(* Logix 5000 AddOnInstructionDefinition export Banner_Q5X_Jam_Param_v4; software revision 33.00 *)

TYPE Banner_BDC_v4 :   // UDT that covers all of the data for BDC options.
STRUCT
   SP1 : DINT;
   SP2 : DINT;   // In FGS, defines the second switching point. Other modes do not use this parameter.
   Switchpoint_Logic : SINT;   // 0 = Light Operate, 1 = Dark Operate
   BDC_Mode : INT;   // 132 = Jam Retroreflective, 133 = Jam Background Suppression
   Hysteresis : INT;   // Hysteresis value for the switchpoint. A value of 0 will result in automatically calculated hysteresis
   Delay_Mode : SINT;   // 0 = Disabled, 1= On-Off Delay, 2 = Oneshot, 3 = Totalizer
   Delay_Time_1 : DINT;   // 0 to 90000
   Delay_Time_2 : DINT;   // 0 to 90000
   BGS_Teach_Offset_Mode : SINT;   // 0 = Auto, 1 = User Selected
   FGS_Window_Size_Mode : SINT;   // 0 = Auto, 1 = User Selected
   User_Teach_Offset : INT;   // User selected teach offset. In FGS or BGS mode this value can be either positive or negative. In BGS mode, this mode must be set to 0 if the Teach Offset Mode is set to Auto. In all other teach modes this value must be written as 0.
   FGS_User_Window_Size : INT;   // In FGS mode this will set the size of the window for a teach. If teach offest mode is set to Auto, this value must be written as 0. In all other teach modes this value must be set to 0.
   Teach_Minimum_Moving_Range : DINT;   // Teach minimum moving range.
   Teach_Jam_Detection_Response_Time : DINT;   // Teach Jam detection response time.
   BDC_AutoThresholding : SINT;   // 0 = On, 1 = Off, 2 = High Speed. Set the auto-thresholding mode (dual teach mode only).
END_STRUCT
END_TYPE

TYPE Banner_IOL_Port_v4 :   // UDT that has all of the data items necessary to communicate with a specific Port on a IO-Link Master
STRUCT
   Port_Controlled : INT;   // Each bit represents a port on an IO-Link Master. Set to 1 to tell AOI to control that port.
   Port_Activate : INT;   // Each bit represents a port on an IO-Link Master. When ON that port will process any commands in queue.
   Port_Read : INT;   // Each bit represents a port on an IO-Link Master. Used to determine when device AOI has requested a Read command.
   Port_Write : INT;   // Each bit represents a port on an IO-Link Master. Used to determine when device AOI has requested a Write command.
   Port_RW_Complete : INT;   // Each bit represents a port on an IO-Link Master. Tells device AOI that Read or Write request has been completed.
   Port_Device_Read : INT;
   Data_Transfer : SINT[190];   // Array to transfer data from IO-Master to device AOIs.
END_STRUCT
END_TYPE

TYPE Banner_Q5X_Jam_RD_v4 :   // UDT that stores the Write Data for a Q5X.
STRUCT
   Master_Cycle_Time : INT;
   Min_Cycle_Time : INT;
   M_Sequence_Capability : INT;
   IO_Link_Version_ID : INT;
   Process_Data_Input_Length : INT;
   Process_Data_Output_Length : INT;
   Combined_Vendor_ID : DINT;   // IO-Link Vendor ID
   Vendor_ID1 : INT;
   Vendor_ID2 : INT;
   Combined_Device_ID : DINT;   // IO-Link Device ID
   Device_ID1 : INT;
   Device_ID2 : INT;
   Device_ID3 : INT;
   Serial_Number : STRING;
   Teach_State : SINT;
   SP1_TP1 : SINT;
   SP1_TP2 : SINT;
   Measurement_1 : DINT;
   Excess_Gain : DINT;   // Amount of single measured over the minimum threshold.
   Stability : SINT;   // 0 = No target exists, 1 = Marginal or multiple peaks, 2 = Stable
   Multiple_Peak_State : SINT;   // 0 = Multiple peaks not present, 1 = Multiple peaks present
   Emitter_Status : SINT;   // 0 = Active, 1 = Inactive
   Laser_Fault_Status : SINT;   // 0 = No Fault, 1 = Fault Present
   BDC1_Totalizer_Counts : DINT;
   BDC2_Totalizer_Counts : DINT;
   All_Time_Run_Time : DINT;   // Read only counter that tracks the total time sensor has been running since manufacture. Value in Hours.
   Display : STRING;   // Last Display information
END_STRUCT
END_TYPE

TYPE Banner_Q5X_Jam_v4 :   // All of the parameters for a Q5X.
STRUCT
   Initial_Global_Read : BOOL;   // Determines if all of the IO-Link data has been read into the PLC yet
   Command : INT;   // Value placed in here will activate a read or write to a specifc IO-Link Index
   Read : Banner_Q5X_Jam_RD_v4;   // Read Only Data
   Write : Banner_Q5X_Jam_WD_v4;   // Write Data
   Archive : Banner_Q5X_Jam_WD_v4;   // Archive Data
   Reset : BOOL;   // Resets AOI. This will force a complete parameter read of the sensor.
END_STRUCT
END_TYPE

TYPE Banner_Q5X_Jam_WD_v4 :   // UDT that stores the Write Data for a Q5X.
STRUCT
   System_Command : INT;   // See IODD file for list of commands that can be activated via the System Command interface
   Parameter_Access_Lock : SINT;   // Write access to all parameters is prohibited while value is 1. Only this parameter can be adjusted when value is 1.
   Data_Storage_Lock : SINT;   // Automatic data storage is disabled when this value is equal to 1. Read access is not affected.
   Local_Parameterization_Lock : SINT;   // Parameterization via local control elements on device is disabled.
   Local_User_Interface_Lock : SINT;   // Operation of local user interface is disabled.
   Teach_in_Channel : SINT;   // 0 = Default, 1 = BDC1, 2 = BDC2
   BDC : Banner_BDC_v4[3];
   Response_Speed : SINT;   // 2 = 15ms, 3 = 25ms, 4 = 50ms
   Gain : SINT;   // 0 = High excess gain mode, 1 = Standard excess gain mode
   Secondary_Output_Mode : SINT;   // 0 = Remote Teach Input, 1 = Laser On, 2 = Master, 3 = Slave, 4 = Complementary Output, 5 = Laser Off, 6 = Pulse Freq Modulation, 7 = Independent Output
   Zero_Reference_Location : SINT;   // 0 = Near, 1 = Far
   Shift_Zero_after_Teach : SINT;   // 0 = Off, 1 = On
   Display_Read : SINT;   // 0 = On, 1 = On Inverted, 2 = Off, 3 = Off Inverted
   Pushbutton_Lockout : SINT;   // 0 = No Lockout, 1 = Pushbuttons Locked, 2 = Operator Lockout
   Output_Polarity : SINT;   // 0 = Default, 1 = PNP, 2 = NPN
   IOL_Filter_Time : INT;   // Time to average IOl process data measurement between updates
   Include_Binary : SINT;   // 0 = Include, 1 = Don't Include
   Measurement_1 : SINT;   // 0 = Disabled, 1 = Excess Gain, 2 = Excess Gain / 10
   Measurement_2 : SINT;   // 0 = Disabled, 1 = Distance Value, 2 = Displayed Distance, 3 = Channel 2 Dual Mode Percent
   Resettable_Run_Time : DINT;
   PFM_Near : DINT;   // 100 to 45000 in Hz
   PFM_Far : DINT;   // 100 to 45000 in Hz
   All_Time_Run_Time_Event_Time : DINT;
   Resettable_Run_Time_Event_Time : DINT;
END_STRUCT
END_TYPE

ADD_ON_INSTRUCTION Banner_Q5X_Jam_Param_v4   (* revision 4.0, vendor Banner Engineering *)
// AOI to read and write parameter data to an IO-Link Q5X.
VAR_IN_OUT
   Q5X : Banner_Q5X_Jam_v4; {required}
   Port_Data : Banner_IOL_Port_v4; {required}
END_VAR
VAR_INPUT
   Port : DINT; {required}
END_VAR
VAR
   Local_Control : DINT; {access None}
   Global_Read_Command_Value : INT; {access None}
   Global_Write_Command_Value : INT; {access None}
   Command_Being_Processed : BOOL; {access None}
   Update_Archive : BOOL; {access None}
   Index_Write_Inprocess : INT; {access None}
   Index_Write_Control : INT; {access None}
   Inprocess_Index : DINT; {access None}
END_VAR

ROUTINE Logic   (* ladder *)
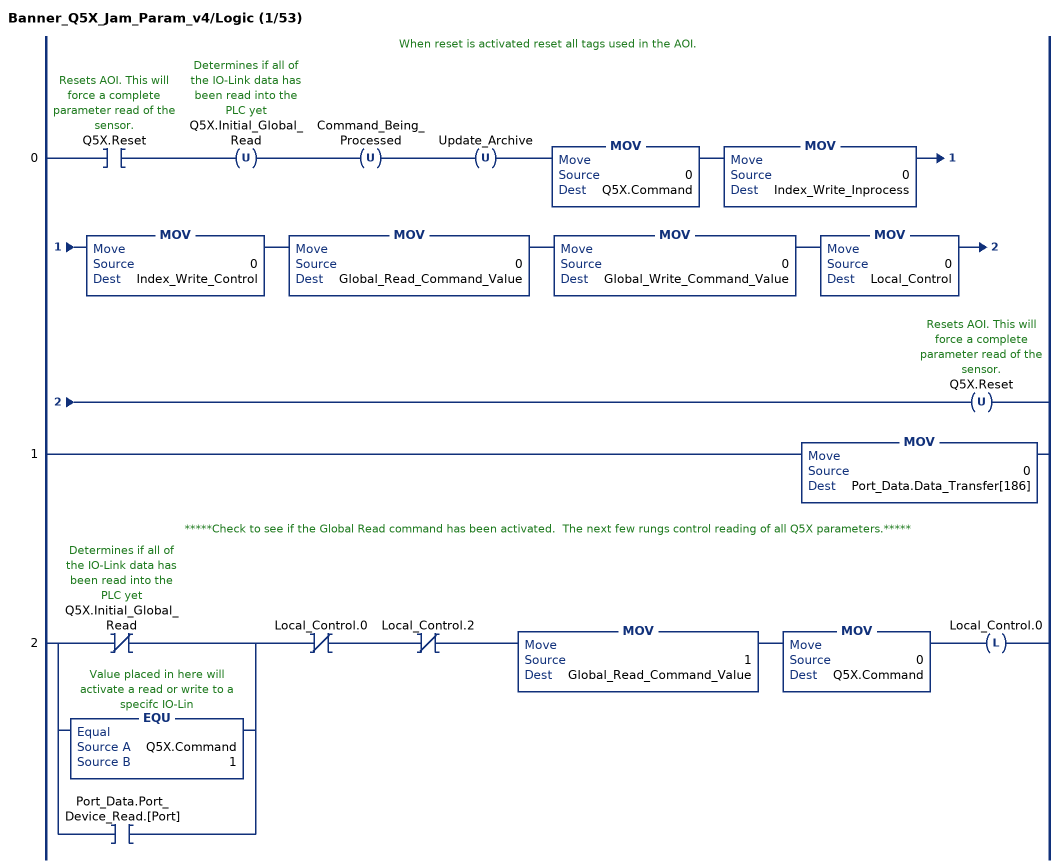
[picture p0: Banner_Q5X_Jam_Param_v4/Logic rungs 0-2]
   // When reset is activated reset all tags used in the AOI.
   0: XIC(Q5X.Reset)OTU(Q5X.Initial_Global_Read)OTU(Command_Being_Processed)OTU(Update_Archive)MOV(0,Q5X.Command)MOV(0,Index_Write_Inprocess)MOV(0,Index_Write_Control)MOV(0,Global_Read_Command_Value)MOV(0,Global_Write_Command_Value)MOV(0,Local_Control)OTU(Q5X.Reset);
   1: MOV(0,Port_Data.Data_Transfer[186]);
   // *****Check to see if the Global Read command has been activated.  The next few rungs control reading of all Q5X parameters.*****
   2: [XIO(Q5X.Initial_Global_Read) ,EQU(Q5X.Command,1) ,XIC(Port_Data.Port_Device_Read.[Port]) ]XIO(Local_Control.0)XIO(Local_Control.2)MOV(1,Global_Read_Command_Value)MOV(0,Q5X.Command)OTL(Local_Control.0);
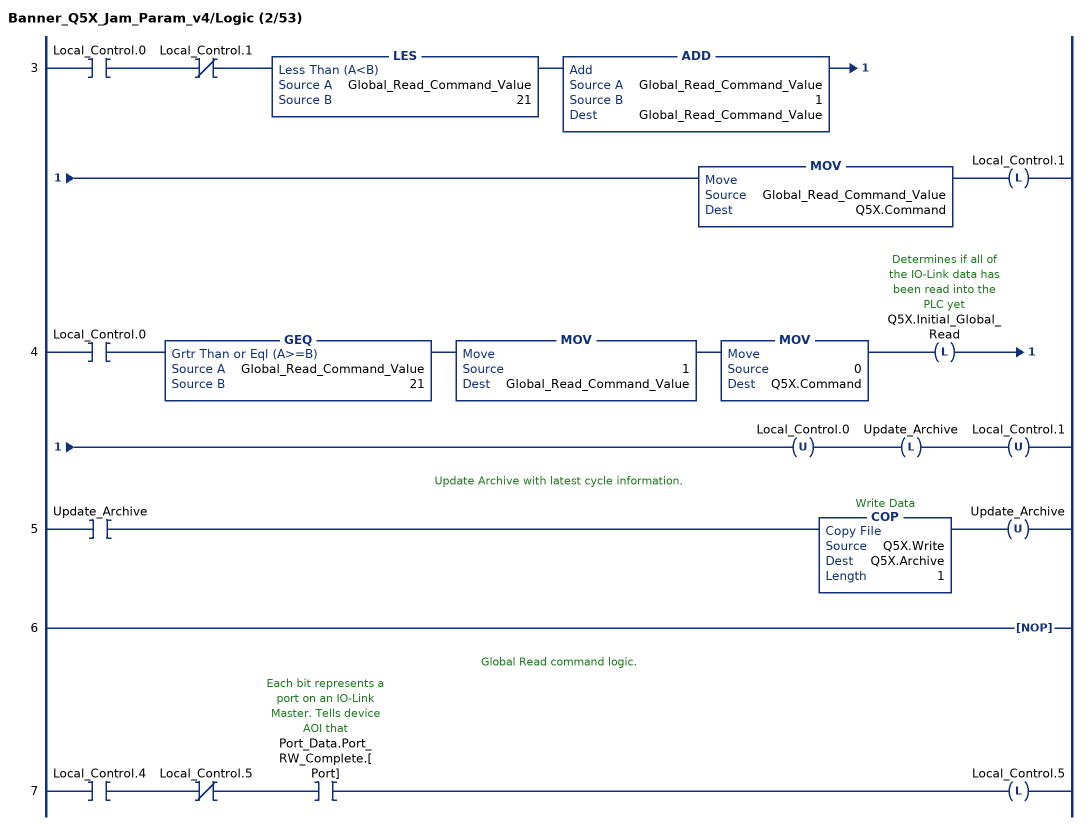
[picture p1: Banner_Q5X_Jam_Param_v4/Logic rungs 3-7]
   3: XIC(Local_Control.0)XIO(Local_Control.1)LES(Global_Read_Command_Value,21)ADD(Global_Read_Command_Value,1,Global_Read_Command_Value)MOV(Global_Read_Command_Value,Q5X.Command)OTL(Local_Control.1);
   4: XIC(Local_Control.0)GEQ(Global_Read_Command_Value,21)MOV(1,Global_Read_Command_Value)MOV(0,Q5X.Command)OTL(Q5X.Initial_Global_Read)OTU(Local_Control.0)OTL(Update_Archive)OTU(Local_Control.1);
   // Update Archive with latest cycle information.
   5: XIC(Update_Archive)COP(Q5X.Write,Q5X.Archive,1)OTU(Update_Archive);
   6: NOP();
   // Global Read command logic.
   7: XIC(Local_Control.4)XIO(Local_Control.5)XIC(Port_Data.Port_RW_Complete.[Port])OTL(Local_Control.5);
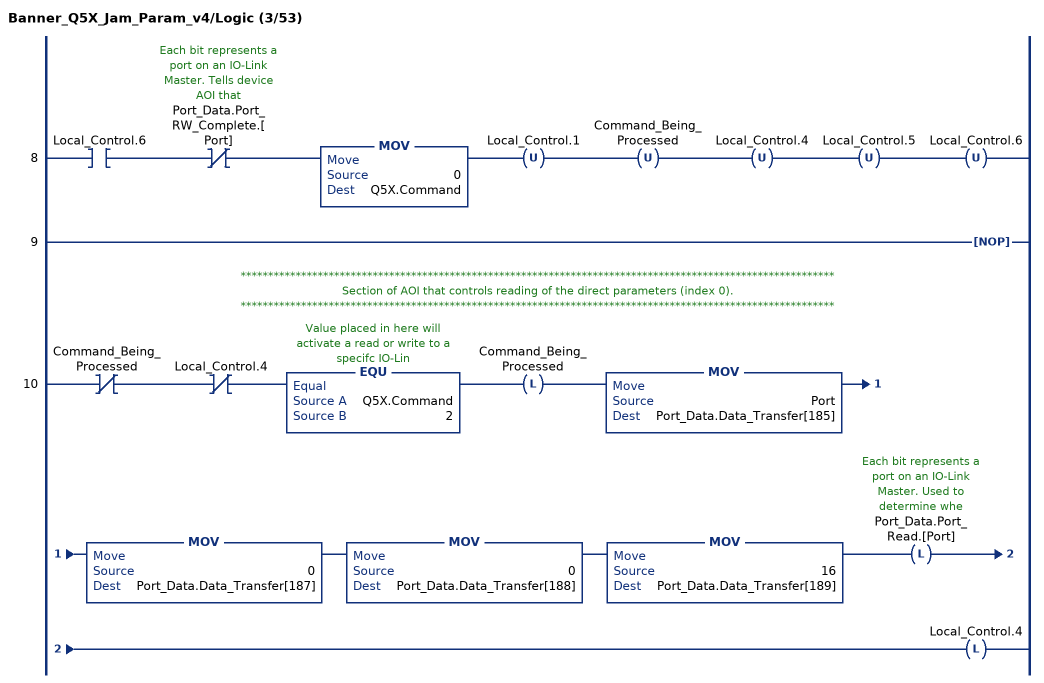
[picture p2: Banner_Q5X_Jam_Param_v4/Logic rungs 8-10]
   8: XIC(Local_Control.6)XIO(Port_Data.Port_RW_Complete.[Port])MOV(0,Q5X.Command)OTU(Local_Control.1)OTU(Command_Being_Processed)OTU(Local_Control.4)OTU(Local_Control.5)OTU(Local_Control.6);
   9: NOP();
   // ************************************************************************************************************
   // Section of AOI that controls reading of the direct parameters (index 0).
   // ************************************************************************************************************
   10: XIO(Command_Being_Processed)XIO(Local_Control.4)EQU(Q5X.Command,2)OTL(Command_Being_Processed)MOV(Port,Port_Data.Data_Transfer[185])MOV(0,Port_Data.Data_Transfer[187])MOV(0,Port_Data.Data_Transfer[188])MOV(16,Port_Data.Data_Transfer[189])OTL(Port_Data.Port_Read.[Port])OTL(Local_Control.4);
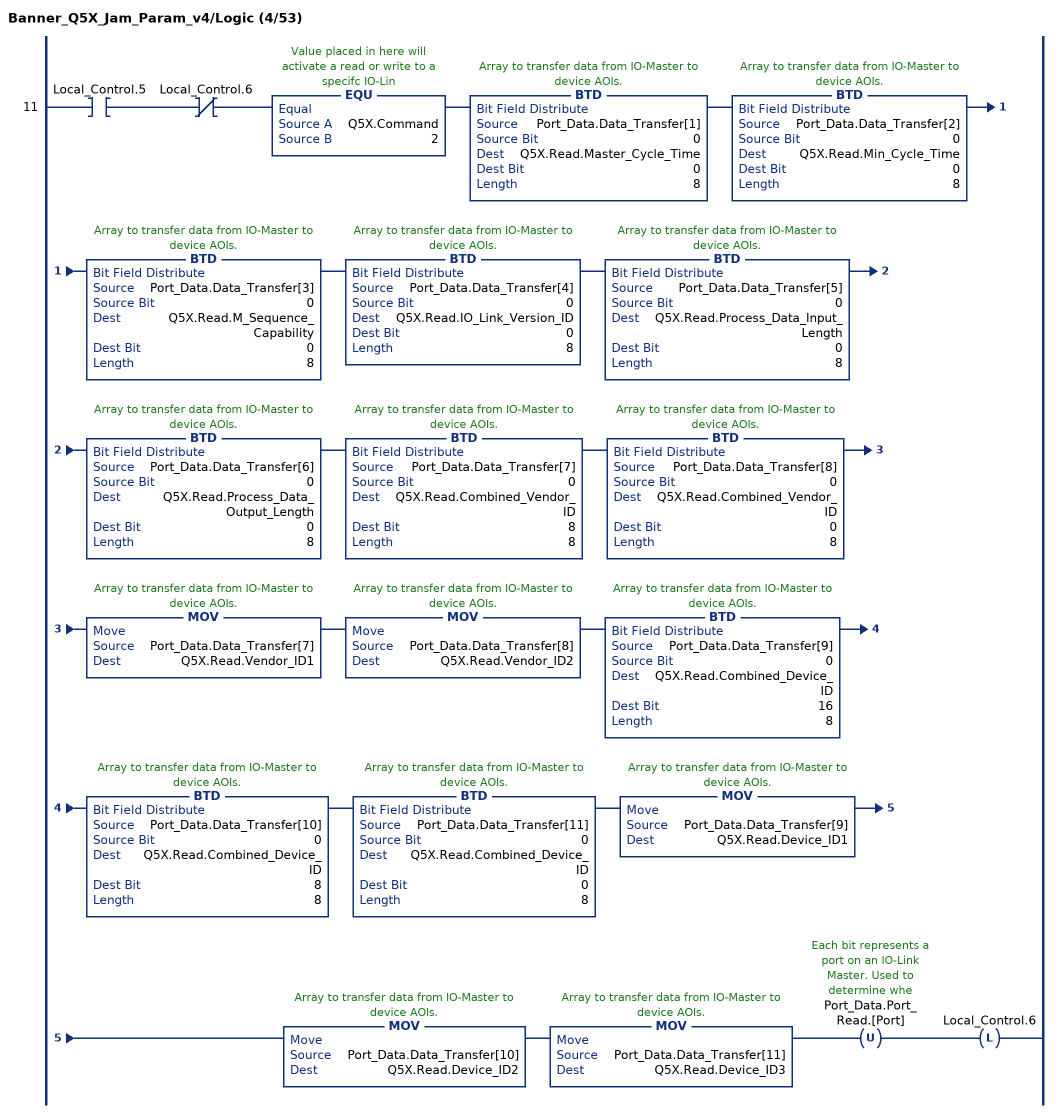
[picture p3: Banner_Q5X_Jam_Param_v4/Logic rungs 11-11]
   11: XIC(Local_Control.5)XIO(Local_Control.6)EQU(Q5X.Command,2)BTD(Port_Data.Data_Transfer[1],0,Q5X.Read.Master_Cycle_Time,0,8)BTD(Port_Data.Data_Transfer[2],0,Q5X.Read.Min_Cycle_Time,0,8)BTD(Port_Data.Data_Transfer[3],0,Q5X.Read.M_Sequence_Capability,0,8)BTD(Port_Data.Data_Transfer[4],0,Q5X.Read.IO_Link_Version_ID,0,8)BTD(Port_Data.Data_Transfer[5],0,Q5X.Read.Process_Data_Input_Length,0,8)BTD(Port_Data.Data_Transfer[6],0,Q5X.Read.Process_Data_Output_Length,0,8)BTD(Port_Data.Data_Transfer[7],0,Q5X.Read.Combined_Vendor_ID,8,8)BTD(Port_Data.Data_Transfer[8],0,Q5X.Read.Combined_Vendor_ID,0,8)MOV(Port_Data.Data_Transfer[7],Q5X.Read.Vendor_ID1)MOV(Port_Data.Data_Transfer[8],Q5X.Read.Vendor_ID2)BTD(Port_Data.Data_Transfer[9],0,Q5X.Read.Combined_Device_ID,16,8)BTD(Port_Data.Data_Transfer[10],0,Q5X.Read.Combined_Device_ID,8,8)BTD(Port_Data.Data_Transfer[11],0,Q5X.Read.Combined_Device_ID,0,8)MOV(Port_Data.Data_Transfer[9],Q5X.Read.Device_ID1)MOV(Port_Data.Data_Transfer[10],Q5X.Read.Device_ID2)MOV(Port_Data.Data_Transfer[11],Q5X.Read.Device_ID3)OTU(Port_Data.Port_Read.[Port])OTL(Local_Control.6);
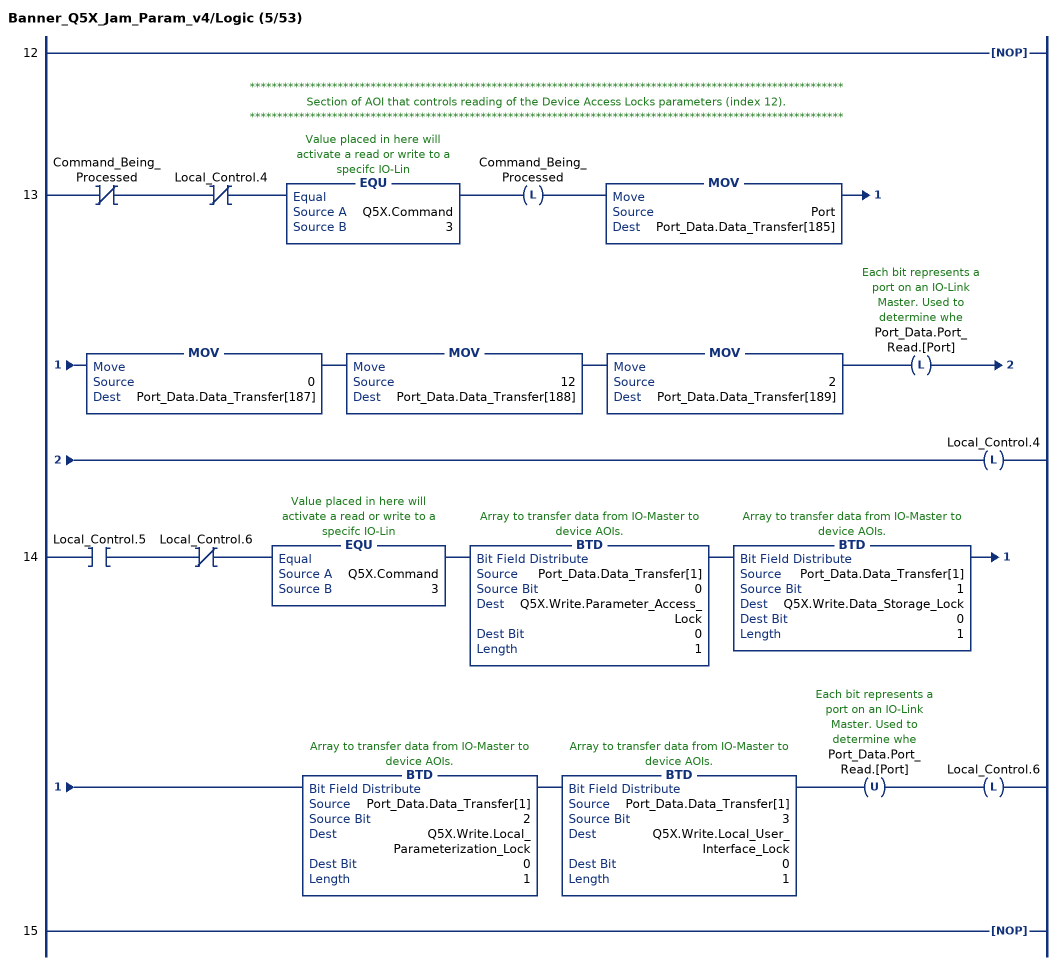
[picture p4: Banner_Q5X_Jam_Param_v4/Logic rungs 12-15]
   12: NOP();
   // ************************************************************************************************************
   // Section of AOI that controls reading of the Device Access Locks parameters (index 12).
   // ************************************************************************************************************
   13: XIO(Command_Being_Processed)XIO(Local_Control.4)EQU(Q5X.Command,3)OTL(Command_Being_Processed)MOV(Port,Port_Data.Data_Transfer[185])MOV(0,Port_Data.Data_Transfer[187])MOV(12,Port_Data.Data_Transfer[188])MOV(2,Port_Data.Data_Transfer[189])OTL(Port_Data.Port_Read.[Port])OTL(Local_Control.4);
   14: XIC(Local_Control.5)XIO(Local_Control.6)EQU(Q5X.Command,3)BTD(Port_Data.Data_Transfer[1],0,Q5X.Write.Parameter_Access_Lock,0,1)BTD(Port_Data.Data_Transfer[1],1,Q5X.Write.Data_Storage_Lock,0,1)BTD(Port_Data.Data_Transfer[1],2,Q5X.Write.Local_Parameterization_Lock,0,1)BTD(Port_Data.Data_Transfer[1],3,Q5X.Write.Local_User_Interface_Lock,0,1)OTU(Port_Data.Port_Read.[Port])OTL(Local_Control.6);
   15: NOP();
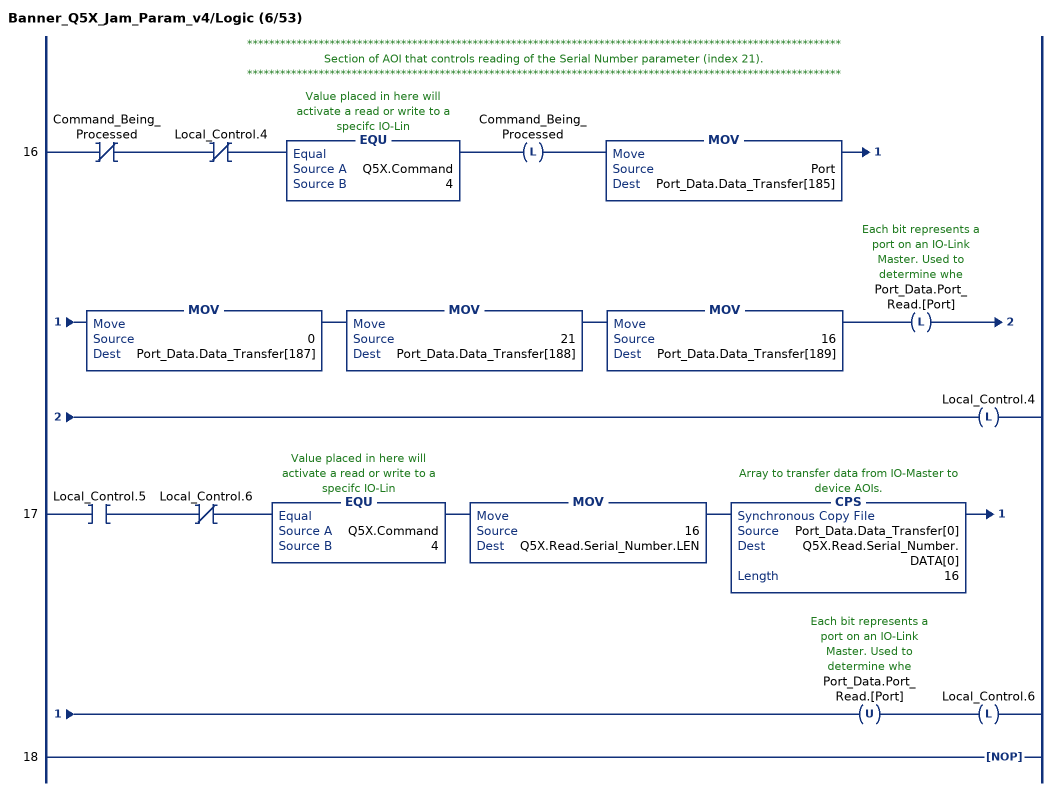
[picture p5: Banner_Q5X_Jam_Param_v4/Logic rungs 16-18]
   // ************************************************************************************************************
   // Section of AOI that controls reading of the Serial Number parameter (index 21).
   // ************************************************************************************************************
   16: XIO(Command_Being_Processed)XIO(Local_Control.4)EQU(Q5X.Command,4)OTL(Command_Being_Processed)MOV(Port,Port_Data.Data_Transfer[185])MOV(0,Port_Data.Data_Transfer[187])MOV(21,Port_Data.Data_Transfer[188])MOV(16,Port_Data.Data_Transfer[189])OTL(Port_Data.Port_Read.[Port])OTL(Local_Control.4);
   17: XIC(Local_Control.5)XIO(Local_Control.6)EQU(Q5X.Command,4)MOV(16,Q5X.Read.Serial_Number.LEN)CPS(Port_Data.Data_Transfer[0],Q5X.Read.Serial_Number.DATA[0],16)OTU(Port_Data.Port_Read.[Port])OTL(Local_Control.6);
   18: NOP();
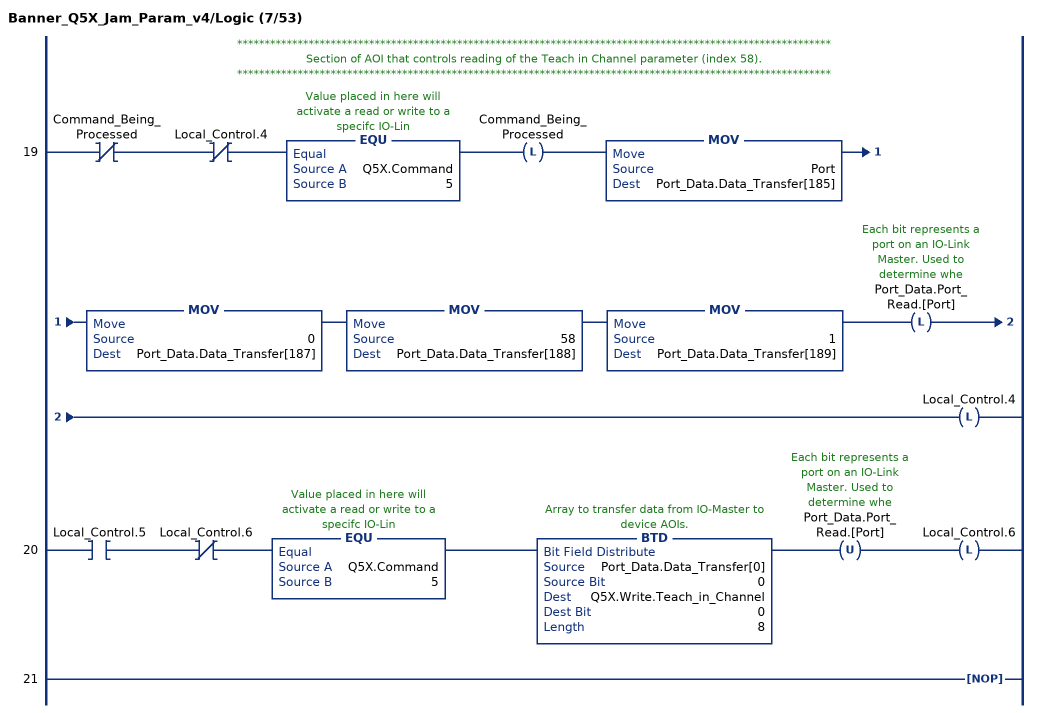
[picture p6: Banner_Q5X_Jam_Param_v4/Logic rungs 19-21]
   // ************************************************************************************************************
   // Section of AOI that controls reading of the Teach in Channel parameter (index 58).
   // ************************************************************************************************************
   19: XIO(Command_Being_Processed)XIO(Local_Control.4)EQU(Q5X.Command,5)OTL(Command_Being_Processed)MOV(Port,Port_Data.Data_Transfer[185])MOV(0,Port_Data.Data_Transfer[187])MOV(58,Port_Data.Data_Transfer[188])MOV(1,Port_Data.Data_Transfer[189])OTL(Port_Data.Port_Read.[Port])OTL(Local_Control.4);
   20: XIC(Local_Control.5)XIO(Local_Control.6)EQU(Q5X.Command,5)BTD(Port_Data.Data_Transfer[0],0,Q5X.Write.Teach_in_Channel,0,8)OTU(Port_Data.Port_Read.[Port])OTL(Local_Control.6);
   21: NOP();
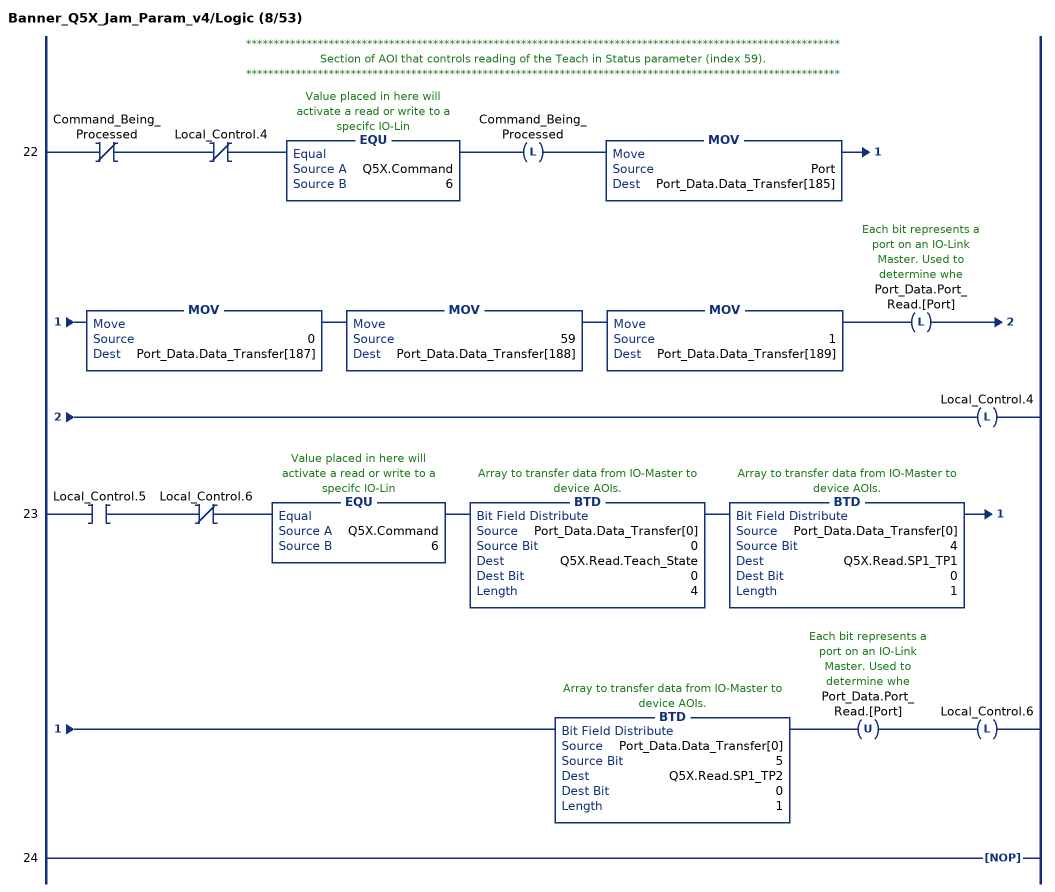
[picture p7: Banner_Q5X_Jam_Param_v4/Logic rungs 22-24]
   // ************************************************************************************************************
   // Section of AOI that controls reading of the Teach in Status parameter (index 59).
   // ************************************************************************************************************
   22: XIO(Command_Being_Processed)XIO(Local_Control.4)EQU(Q5X.Command,6)OTL(Command_Being_Processed)MOV(Port,Port_Data.Data_Transfer[185])MOV(0,Port_Data.Data_Transfer[187])MOV(59,Port_Data.Data_Transfer[188])MOV(1,Port_Data.Data_Transfer[189])OTL(Port_Data.Port_Read.[Port])OTL(Local_Control.4);
   23: XIC(Local_Control.5)XIO(Local_Control.6)EQU(Q5X.Command,6)BTD(Port_Data.Data_Transfer[0],0,Q5X.Read.Teach_State,0,4)BTD(Port_Data.Data_Transfer[0],4,Q5X.Read.SP1_TP1,0,1)BTD(Port_Data.Data_Transfer[0],5,Q5X.Read.SP1_TP2,0,1)OTU(Port_Data.Port_Read.[Port])OTL(Local_Control.6);
   24: NOP();
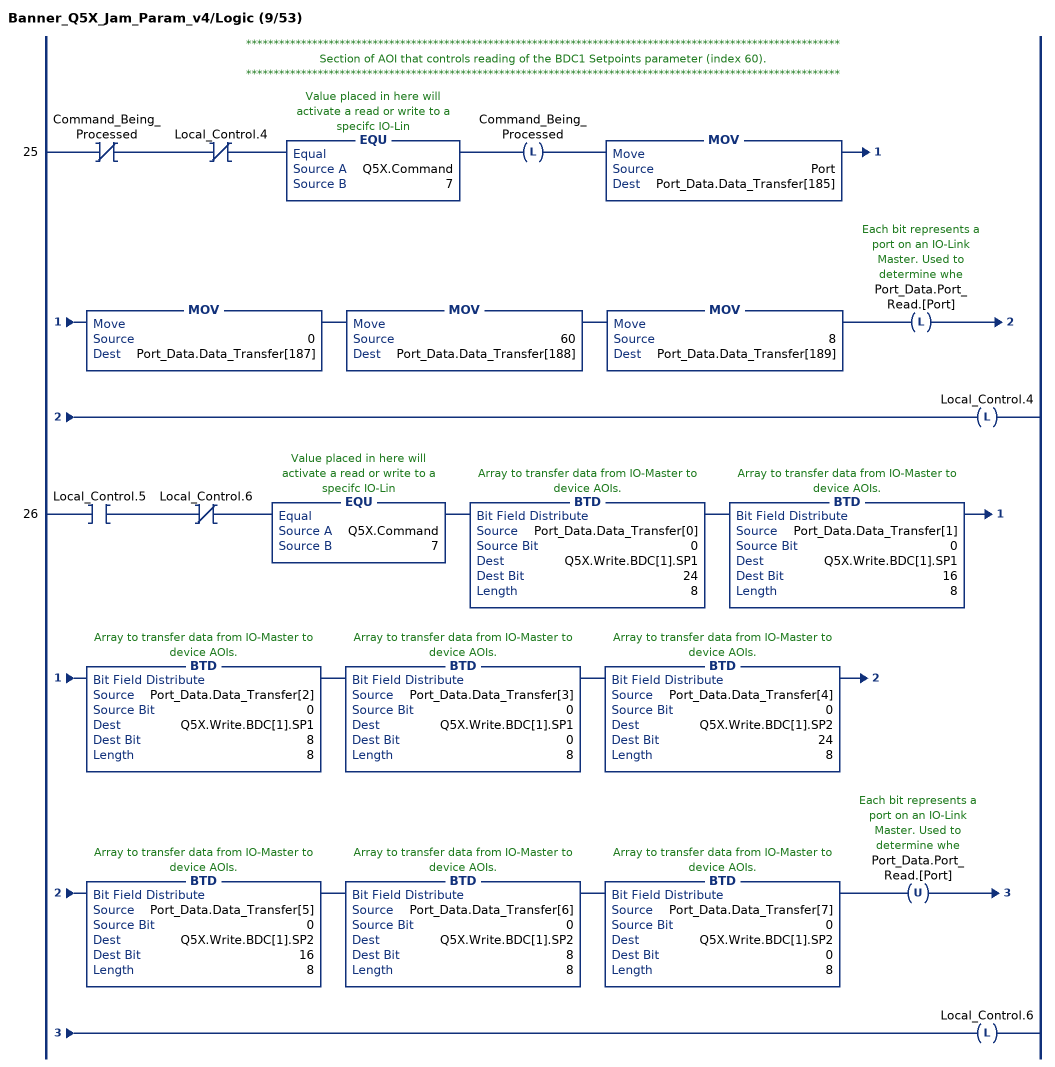
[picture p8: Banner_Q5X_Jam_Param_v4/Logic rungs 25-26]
   // ************************************************************************************************************
   // Section of AOI that controls reading of the BDC1 Setpoints parameter (index 60).
   // ************************************************************************************************************
   25: XIO(Command_Being_Processed)XIO(Local_Control.4)EQU(Q5X.Command,7)OTL(Command_Being_Processed)MOV(Port,Port_Data.Data_Transfer[185])MOV(0,Port_Data.Data_Transfer[187])MOV(60,Port_Data.Data_Transfer[188])MOV(8,Port_Data.Data_Transfer[189])OTL(Port_Data.Port_Read.[Port])OTL(Local_Control.4);
   26: XIC(Local_Control.5)XIO(Local_Control.6)EQU(Q5X.Command,7)BTD(Port_Data.Data_Transfer[0],0,Q5X.Write.BDC[1].SP1,24,8)BTD(Port_Data.Data_Transfer[1],0,Q5X.Write.BDC[1].SP1,16,8)BTD(Port_Data.Data_Transfer[2],0,Q5X.Write.BDC[1].SP1,8,8)BTD(Port_Data.Data_Transfer[3],0,Q5X.Write.BDC[1].SP1,0,8)BTD(Port_Data.Data_Transfer[4],0,Q5X.Write.BDC[1].SP2,24,8)BTD(Port_Data.Data_Transfer[5],0,Q5X.Write.BDC[1].SP2,16,8)BTD(Port_Data.Data_Transfer[6],0,Q5X.Write.BDC[1].SP2,8,8)BTD(Port_Data.Data_Transfer[7],0,Q5X.Write.BDC[1].SP2,0,8)OTU(Port_Data.Port_Read.[Port])OTL(Local_Control.6);
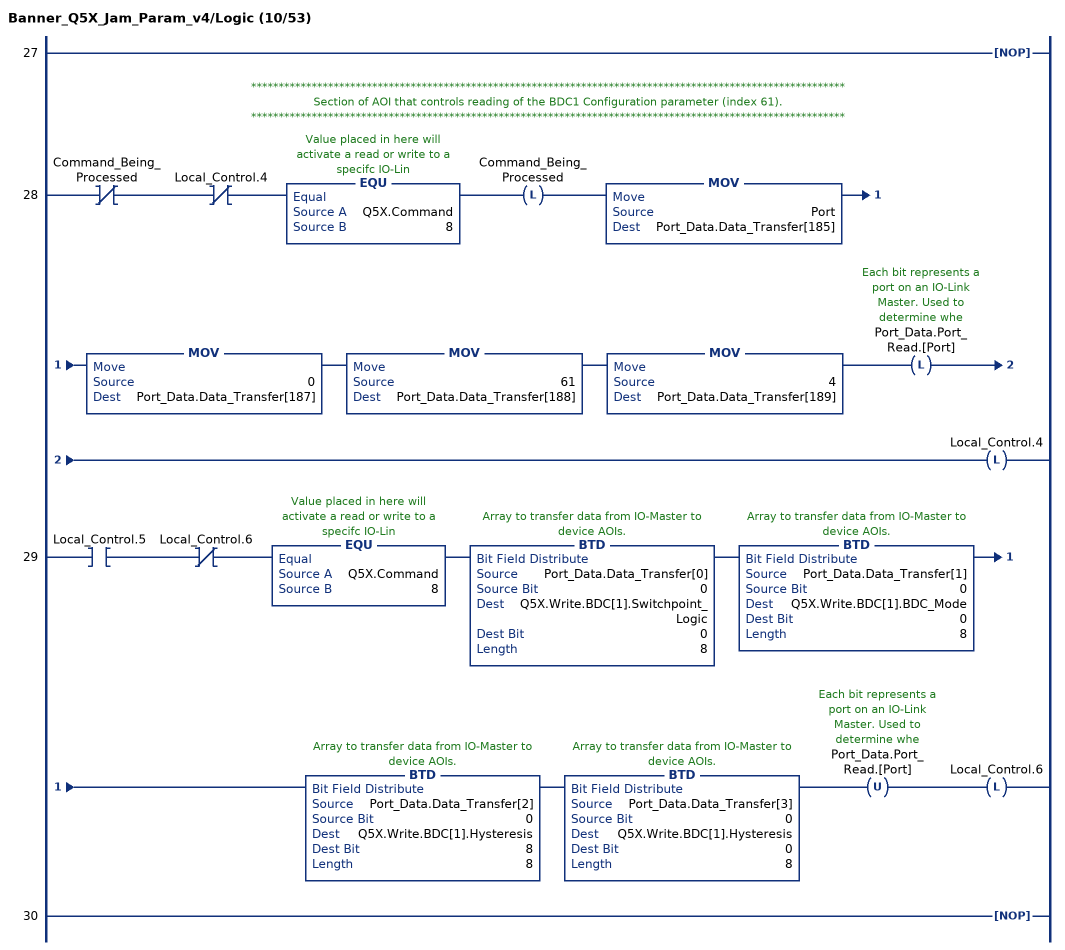
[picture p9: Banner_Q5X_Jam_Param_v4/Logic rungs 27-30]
   27: NOP();
   // ************************************************************************************************************
   // Section of AOI that controls reading of the BDC1 Configuration parameter (index 61).
   // ************************************************************************************************************
   28: XIO(Command_Being_Processed)XIO(Local_Control.4)EQU(Q5X.Command,8)OTL(Command_Being_Processed)MOV(Port,Port_Data.Data_Transfer[185])MOV(0,Port_Data.Data_Transfer[187])MOV(61,Port_Data.Data_Transfer[188])MOV(4,Port_Data.Data_Transfer[189])OTL(Port_Data.Port_Read.[Port])OTL(Local_Control.4);
   29: XIC(Local_Control.5)XIO(Local_Control.6)EQU(Q5X.Command,8)BTD(Port_Data.Data_Transfer[0],0,Q5X.Write.BDC[1].Switchpoint_Logic,0,8)BTD(Port_Data.Data_Transfer[1],0,Q5X.Write.BDC[1].BDC_Mode,0,8)BTD(Port_Data.Data_Transfer[2],0,Q5X.Write.BDC[1].Hysteresis,8,8)BTD(Port_Data.Data_Transfer[3],0,Q5X.Write.BDC[1].Hysteresis,0,8)OTU(Port_Data.Port_Read.[Port])OTL(Local_Control.6);
   30: NOP();
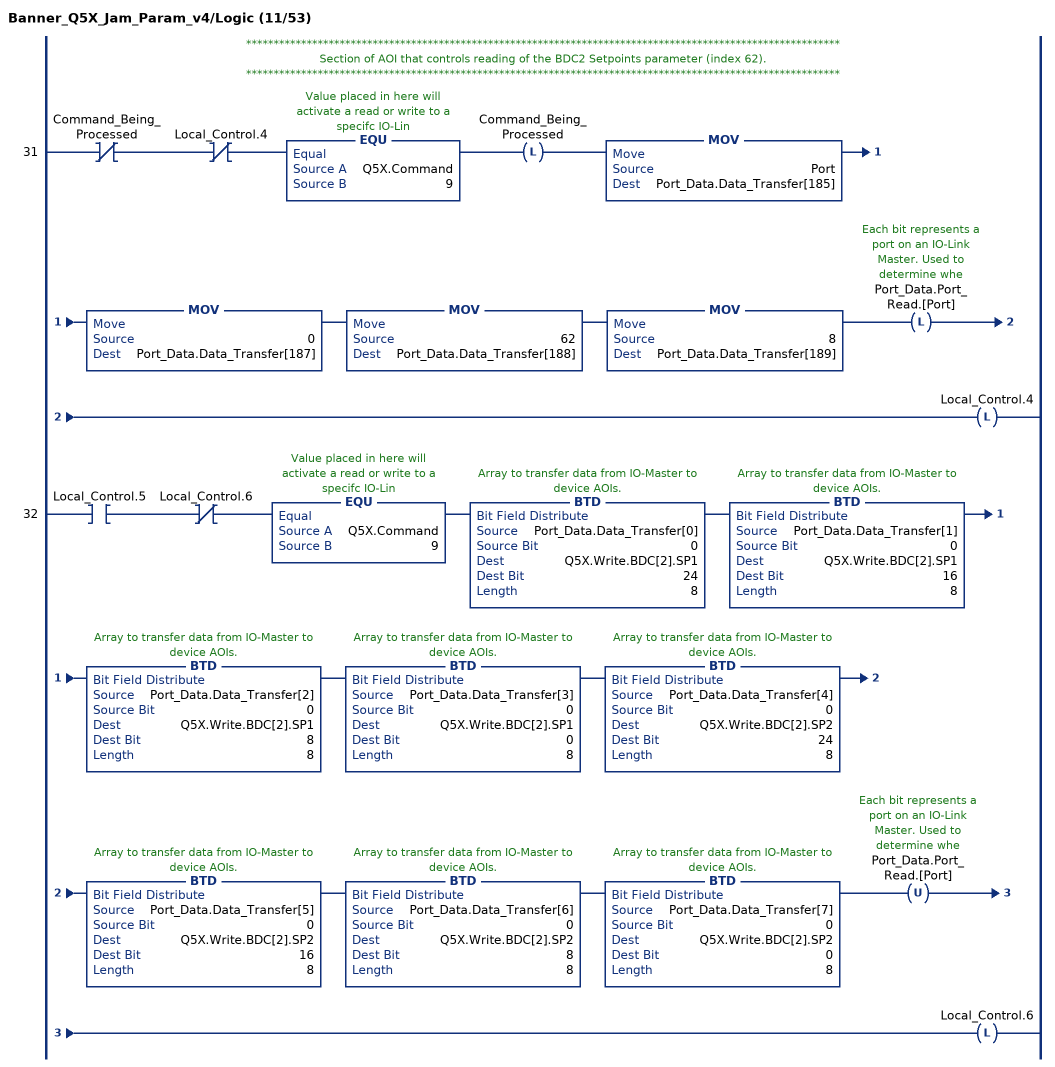
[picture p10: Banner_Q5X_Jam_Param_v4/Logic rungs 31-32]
   // ************************************************************************************************************
   // Section of AOI that controls reading of the BDC2 Setpoints parameter (index 62).
   // ************************************************************************************************************
   31: XIO(Command_Being_Processed)XIO(Local_Control.4)EQU(Q5X.Command,9)OTL(Command_Being_Processed)MOV(Port,Port_Data.Data_Transfer[185])MOV(0,Port_Data.Data_Transfer[187])MOV(62,Port_Data.Data_Transfer[188])MOV(8,Port_Data.Data_Transfer[189])OTL(Port_Data.Port_Read.[Port])OTL(Local_Control.4);
   32: XIC(Local_Control.5)XIO(Local_Control.6)EQU(Q5X.Command,9)BTD(Port_Data.Data_Transfer[0],0,Q5X.Write.BDC[2].SP1,24,8)BTD(Port_Data.Data_Transfer[1],0,Q5X.Write.BDC[2].SP1,16,8)BTD(Port_Data.Data_Transfer[2],0,Q5X.Write.BDC[2].SP1,8,8)BTD(Port_Data.Data_Transfer[3],0,Q5X.Write.BDC[2].SP1,0,8)BTD(Port_Data.Data_Transfer[4],0,Q5X.Write.BDC[2].SP2,24,8)BTD(Port_Data.Data_Transfer[5],0,Q5X.Write.BDC[2].SP2,16,8)BTD(Port_Data.Data_Transfer[6],0,Q5X.Write.BDC[2].SP2,8,8)BTD(Port_Data.Data_Transfer[7],0,Q5X.Write.BDC[2].SP2,0,8)OTU(Port_Data.Port_Read.[Port])OTL(Local_Control.6);
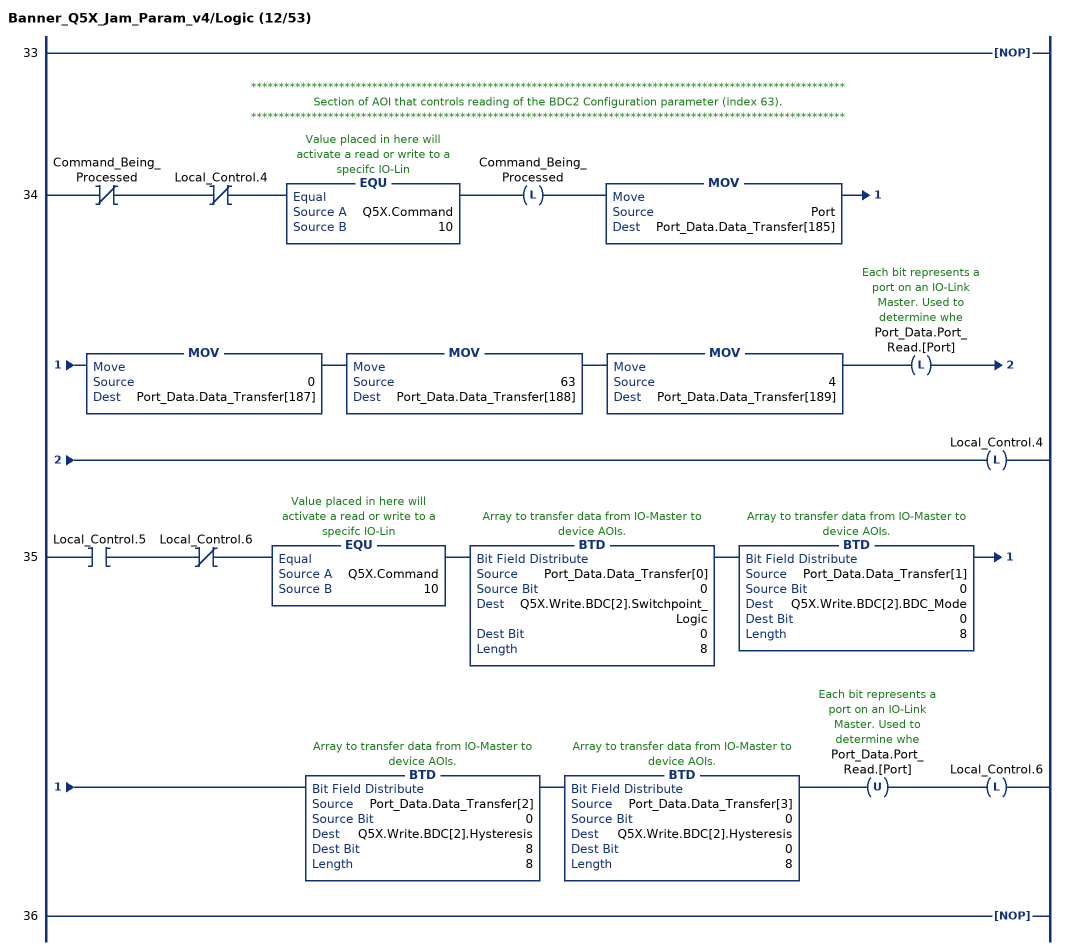
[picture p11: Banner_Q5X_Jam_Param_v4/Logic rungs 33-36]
   33: NOP();
   // ************************************************************************************************************
   // Section of AOI that controls reading of the BDC2 Configuration parameter (index 63).
   // ************************************************************************************************************
   34: XIO(Command_Being_Processed)XIO(Local_Control.4)EQU(Q5X.Command,10)OTL(Command_Being_Processed)MOV(Port,Port_Data.Data_Transfer[185])MOV(0,Port_Data.Data_Transfer[187])MOV(63,Port_Data.Data_Transfer[188])MOV(4,Port_Data.Data_Transfer[189])OTL(Port_Data.Port_Read.[Port])OTL(Local_Control.4);
   35: XIC(Local_Control.5)XIO(Local_Control.6)EQU(Q5X.Command,10)BTD(Port_Data.Data_Transfer[0],0,Q5X.Write.BDC[2].Switchpoint_Logic,0,8)BTD(Port_Data.Data_Transfer[1],0,Q5X.Write.BDC[2].BDC_Mode,0,8)BTD(Port_Data.Data_Transfer[2],0,Q5X.Write.BDC[2].Hysteresis,8,8)BTD(Port_Data.Data_Transfer[3],0,Q5X.Write.BDC[2].Hysteresis,0,8)OTU(Port_Data.Port_Read.[Port])OTL(Local_Control.6);
   36: NOP();
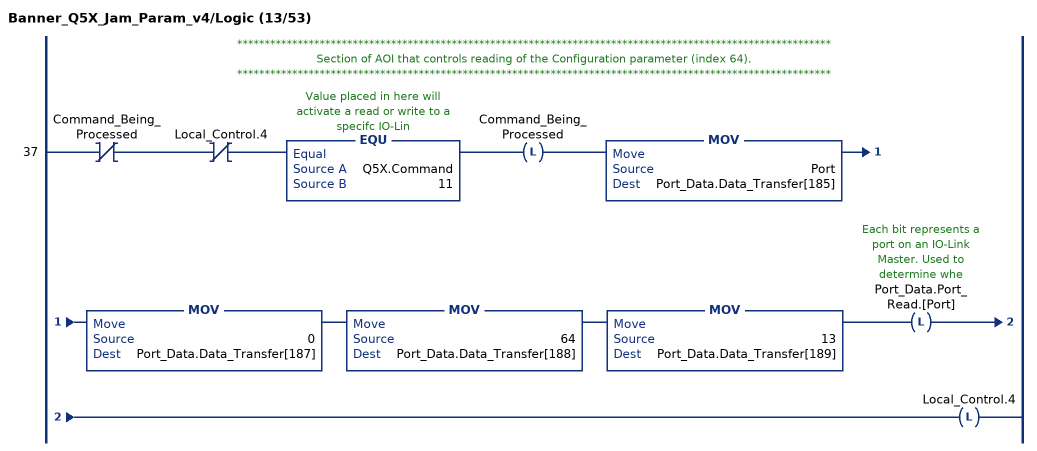
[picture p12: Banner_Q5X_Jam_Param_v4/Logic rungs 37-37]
   // ************************************************************************************************************
   // Section of AOI that controls reading of the Configuration parameter (index 64).
   // ************************************************************************************************************
   37: XIO(Command_Being_Processed)XIO(Local_Control.4)EQU(Q5X.Command,11)OTL(Command_Being_Processed)MOV(Port,Port_Data.Data_Transfer[185])MOV(0,Port_Data.Data_Transfer[187])MOV(64,Port_Data.Data_Transfer[188])MOV(13,Port_Data.Data_Transfer[189])OTL(Port_Data.Port_Read.[Port])OTL(Local_Control.4);
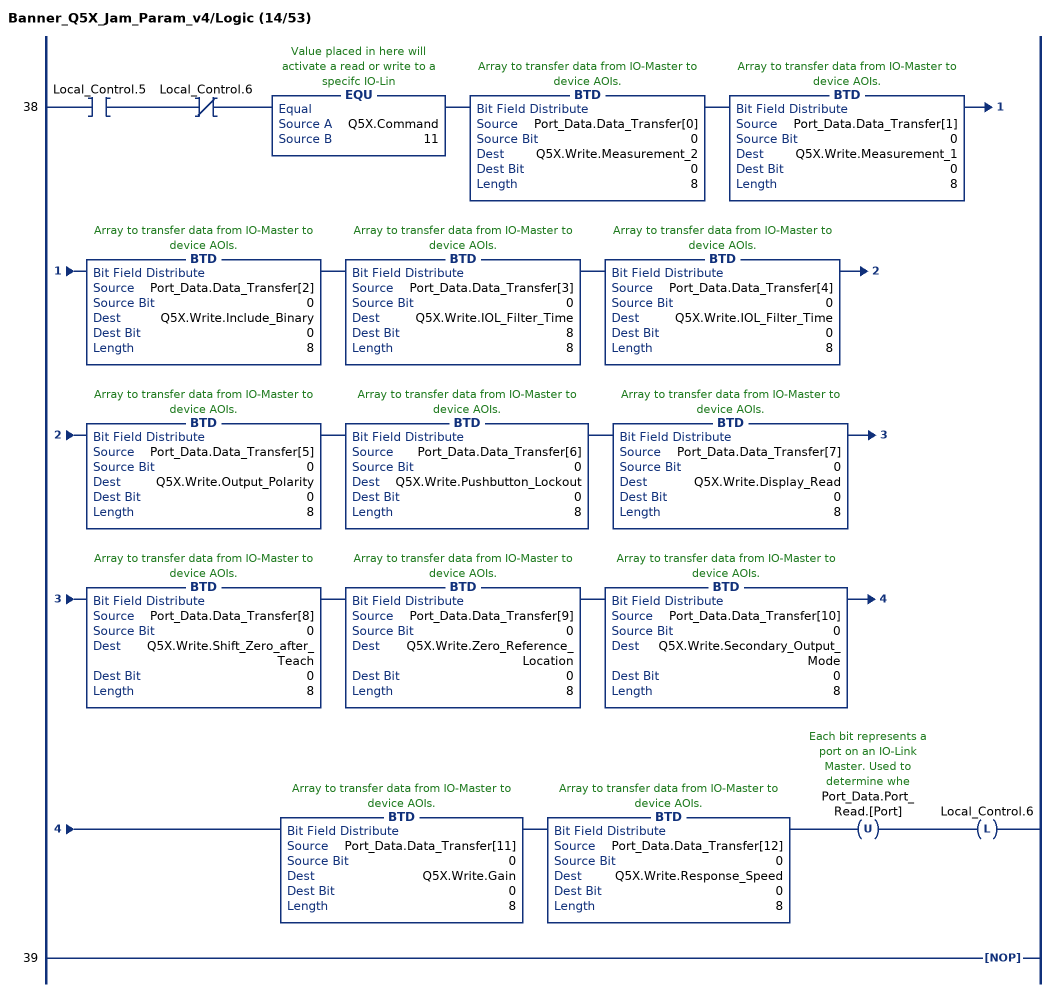
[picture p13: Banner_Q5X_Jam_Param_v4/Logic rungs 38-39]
   38: XIC(Local_Control.5)XIO(Local_Control.6)EQU(Q5X.Command,11)BTD(Port_Data.Data_Transfer[0],0,Q5X.Write.Measurement_2,0,8)BTD(Port_Data.Data_Transfer[1],0,Q5X.Write.Measurement_1,0,8)BTD(Port_Data.Data_Transfer[2],0,Q5X.Write.Include_Binary,0,8)BTD(Port_Data.Data_Transfer[3],0,Q5X.Write.IOL_Filter_Time,8,8)BTD(Port_Data.Data_Transfer[4],0,Q5X.Write.IOL_Filter_Time,0,8)BTD(Port_Data.Data_Transfer[5],0,Q5X.Write.Output_Polarity,0,8)BTD(Port_Data.Data_Transfer[6],0,Q5X.Write.Pushbutton_Lockout,0,8)BTD(Port_Data.Data_Transfer[7],0,Q5X.Write.Display_Read,0,8)BTD(Port_Data.Data_Transfer[8],0,Q5X.Write.Shift_Zero_after_Teach,0,8)BTD(Port_Data.Data_Transfer[9],0,Q5X.Write.Zero_Reference_Location,0,8)BTD(Port_Data.Data_Transfer[10],0,Q5X.Write.Secondary_Output_Mode,0,8)BTD(Port_Data.Data_Transfer[11],0,Q5X.Write.Gain,0,8)BTD(Port_Data.Data_Transfer[12],0,Q5X.Write.Response_Speed,0,8)OTU(Port_Data.Port_Read.[Port])OTL(Local_Control.6);
   39: NOP();
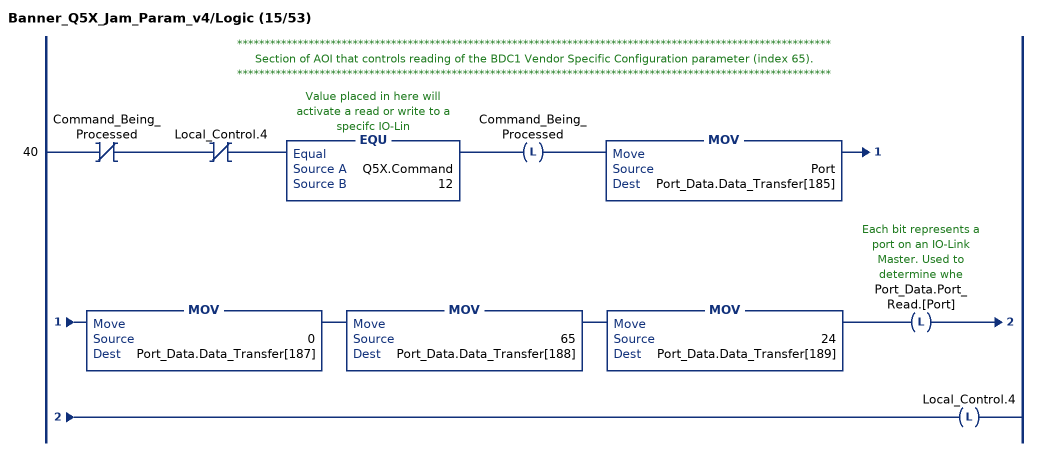
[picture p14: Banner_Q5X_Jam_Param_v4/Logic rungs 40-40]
   // ************************************************************************************************************
   // Section of AOI that controls reading of the BDC1 Vendor Specific Configuration parameter (index 65).
   // ************************************************************************************************************
   40: XIO(Command_Being_Processed)XIO(Local_Control.4)EQU(Q5X.Command,12)OTL(Command_Being_Processed)MOV(Port,Port_Data.Data_Transfer[185])MOV(0,Port_Data.Data_Transfer[187])MOV(65,Port_Data.Data_Transfer[188])MOV(24,Port_Data.Data_Transfer[189])OTL(Port_Data.Port_Read.[Port])OTL(Local_Control.4);
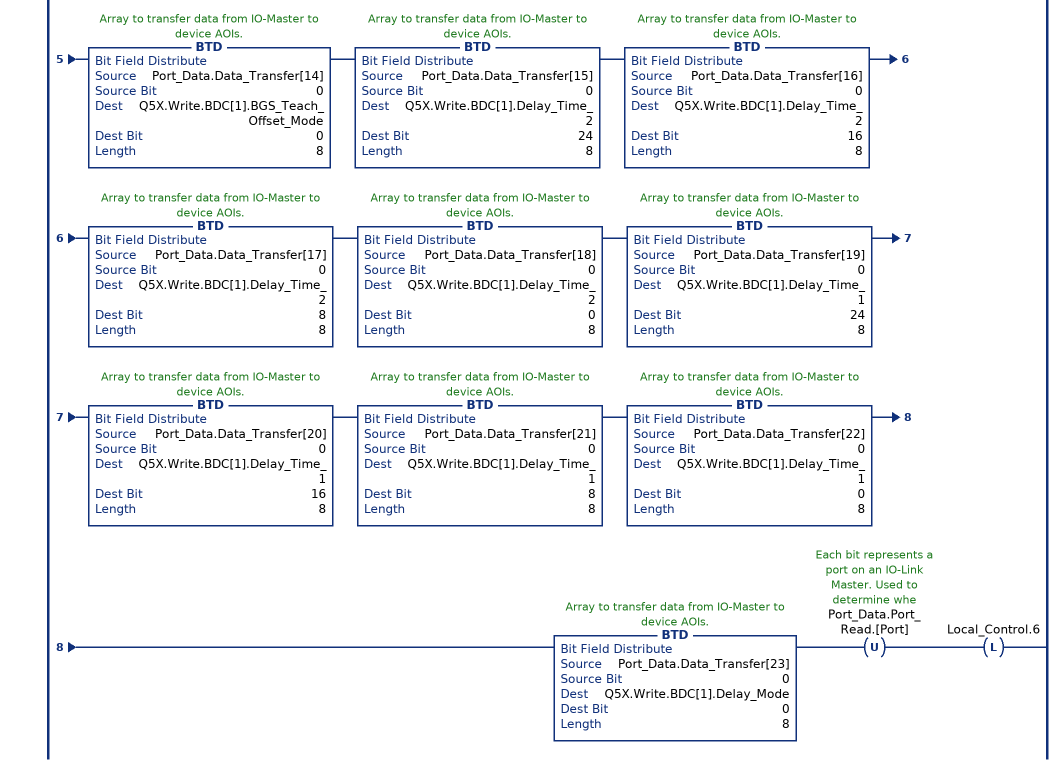
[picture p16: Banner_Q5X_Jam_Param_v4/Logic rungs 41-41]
   41: XIC(Local_Control.5)XIO(Local_Control.6)EQU(Q5X.Command,12)BTD(Port_Data.Data_Transfer[0],0,Q5X.Write.BDC[1].BDC_AutoThresholding,0,8)BTD(Port_Data.Data_Transfer[1],0,Q5X.Write.BDC[1].Teach_Jam_Detection_Response_Time,24,8)BTD(Port_Data.Data_Transfer[2],0,Q5X.Write.BDC[1].Teach_Jam_Detection_Response_Time,16,8)BTD(Port_Data.Data_Transfer[3],0,Q5X.Write.BDC[1].Teach_Jam_Detection_Response_Time,8,8)BTD(Port_Data.Data_Transfer[4],0,Q5X.Write.BDC[1].Teach_Jam_Detection_Response_Time,0,8)BTD(Port_Data.Data_Transfer[5],0,Q5X.Write.BDC[1].Teach_Minimum_Moving_Range,24,8)BTD(Port_Data.Data_Transfer[6],0,Q5X.Write.BDC[1].Teach_Minimum_Moving_Range,16,8)BTD(Port_Data.Data_Transfer[7],0,Q5X.Write.BDC[1].Teach_Minimum_Moving_Range,8,8)BTD(Port_Data.Data_Transfer[8],0,Q5X.Write.BDC[1].Teach_Minimum_Moving_Range,0,8)BTD(Port_Data.Data_Transfer[9],0,Q5X.Write.BDC[1].FGS_User_Window_Size,8,8)BTD(Port_Data.Data_Transfer[10],0,Q5X.Write.BDC[1].FGS_User_Window_Size,0,8)BTD(Port_Data.Data_Transfer[11],0,Q5X.Write.BDC[1].User_Teach_Offset,8,8)BTD(Port_Data.Data_Transfer[12],0,Q5X.Write.BDC[1].User_Teach_Offset,0,8)BTD(Port_Data.Data_Transfer[13],0,Q5X.Write.BDC[1].FGS_Window_Size_Mode,0,8)BTD(Port_Data.Data_Transfer[14],0,Q5X.Write.BDC[1].BGS_Teach_Offset_Mode,0,8)BTD(Port_Data.Data_Transfer[15],0,Q5X.Write.BDC[1].Delay_Time_2,24,8)BTD(Port_Data.Data_Transfer[16],0,Q5X.Write.BDC[1].Delay_Time_2,16,8)BTD(Port_Data.Data_Transfer[17],0,Q5X.Write.BDC[1].Delay_Time_2,8,8)BTD(Port_Data.Data_Transfer[18],0,Q5X.Write.BDC[1].Delay_Time_2,0,8)BTD(Port_Data.Data_Transfer[19],0,Q5X.Write.BDC[1].Delay_Time_1,24,8)BTD(Port_Data.Data_Transfer[20],0,Q5X.Write.BDC[1].Delay_Time_1,16,8)BTD(Port_Data.Data_Transfer[21],0,Q5X.Write.BDC[1].Delay_Time_1,8,8)BTD(Port_Data.Data_Transfer[22],0,Q5X.Write.BDC[1].Delay_Time_1,0,8)BTD(Port_Data.Data_Transfer[23],0,Q5X.Write.BDC[1].Delay_Mode,0,8)OTU(Port_Data.Port_Read.[Port])OTL(Local_Control.6);
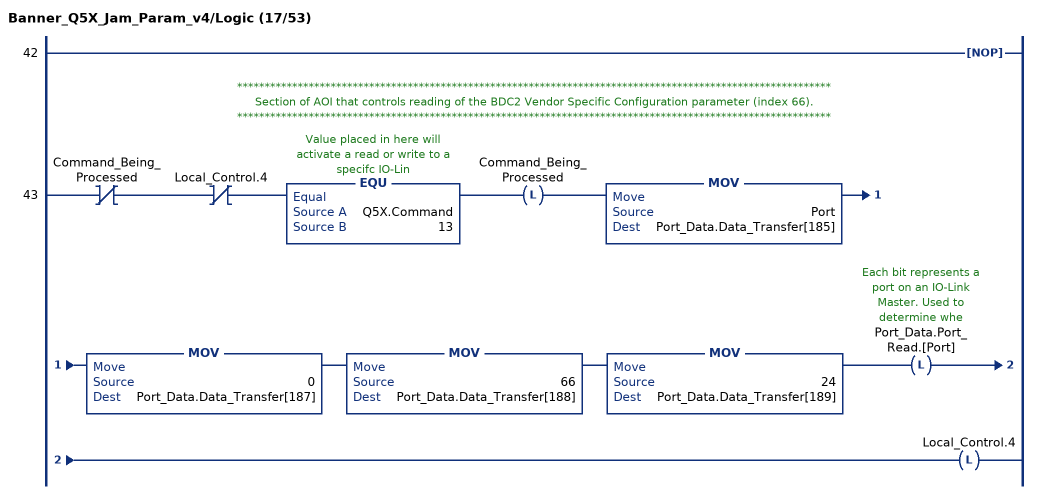
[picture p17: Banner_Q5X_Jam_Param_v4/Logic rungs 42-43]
   42: NOP();
   // ************************************************************************************************************
   // Section of AOI that controls reading of the BDC2 Vendor Specific Configuration parameter (index 66).
   // ************************************************************************************************************
   43: XIO(Command_Being_Processed)XIO(Local_Control.4)EQU(Q5X.Command,13)OTL(Command_Being_Processed)MOV(Port,Port_Data.Data_Transfer[185])MOV(0,Port_Data.Data_Transfer[187])MOV(66,Port_Data.Data_Transfer[188])MOV(24,Port_Data.Data_Transfer[189])OTL(Port_Data.Port_Read.[Port])OTL(Local_Control.4);
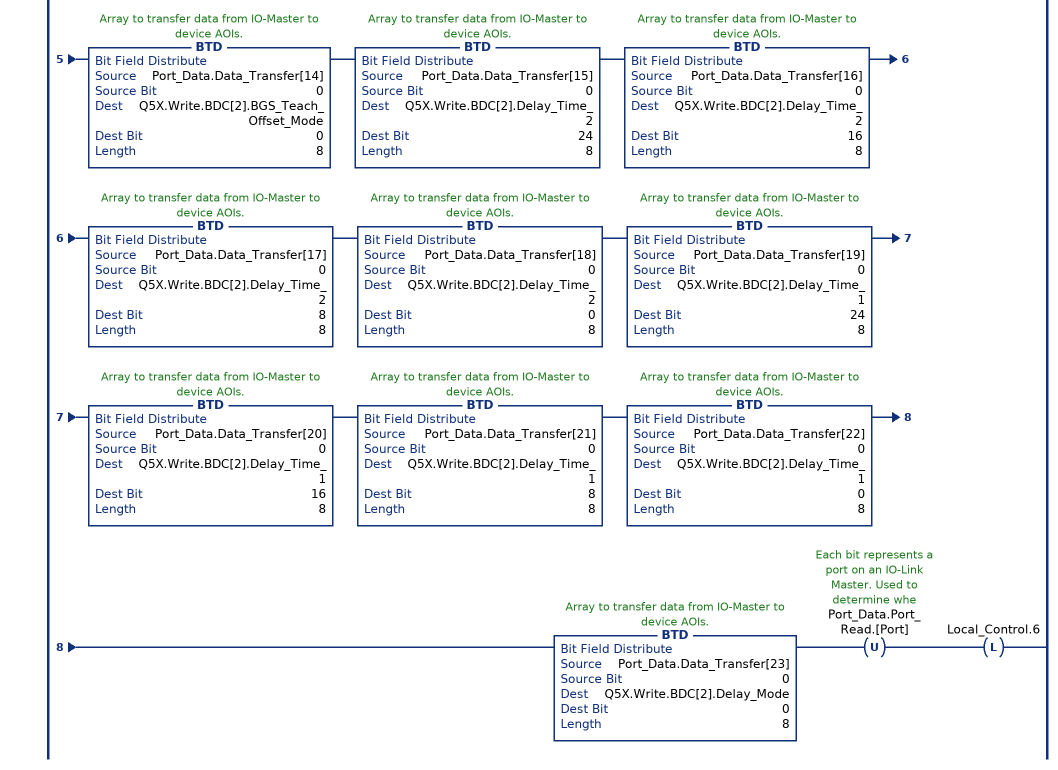
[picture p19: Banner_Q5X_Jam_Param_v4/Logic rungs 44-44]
   44: XIC(Local_Control.5)XIO(Local_Control.6)EQU(Q5X.Command,13)BTD(Port_Data.Data_Transfer[0],0,Q5X.Write.BDC[2].BDC_AutoThresholding,0,8)BTD(Port_Data.Data_Transfer[1],0,Q5X.Write.BDC[2].Teach_Jam_Detection_Response_Time,24,8)BTD(Port_Data.Data_Transfer[2],0,Q5X.Write.BDC[2].Teach_Jam_Detection_Response_Time,16,8)BTD(Port_Data.Data_Transfer[3],0,Q5X.Write.BDC[2].Teach_Jam_Detection_Response_Time,8,8)BTD(Port_Data.Data_Transfer[4],0,Q5X.Write.BDC[2].Teach_Jam_Detection_Response_Time,0,8)BTD(Port_Data.Data_Transfer[5],0,Q5X.Write.BDC[2].Teach_Minimum_Moving_Range,24,8)BTD(Port_Data.Data_Transfer[6],0,Q5X.Write.BDC[2].Teach_Minimum_Moving_Range,16,8)BTD(Port_Data.Data_Transfer[7],0,Q5X.Write.BDC[2].Teach_Minimum_Moving_Range,8,8)BTD(Port_Data.Data_Transfer[8],0,Q5X.Write.BDC[2].Teach_Minimum_Moving_Range,0,8)BTD(Port_Data.Data_Transfer[9],0,Q5X.Write.BDC[2].FGS_User_Window_Size,8,8)BTD(Port_Data.Data_Transfer[10],0,Q5X.Write.BDC[2].FGS_User_Window_Size,0,8)BTD(Port_Data.Data_Transfer[11],0,Q5X.Write.BDC[2].User_Teach_Offset,8,8)BTD(Port_Data.Data_Transfer[12],0,Q5X.Write.BDC[2].User_Teach_Offset,0,8)BTD(Port_Data.Data_Transfer[13],0,Q5X.Write.BDC[2].FGS_Window_Size_Mode,0,8)BTD(Port_Data.Data_Transfer[14],0,Q5X.Write.BDC[2].BGS_Teach_Offset_Mode,0,8)BTD(Port_Data.Data_Transfer[15],0,Q5X.Write.BDC[2].Delay_Time_2,24,8)BTD(Port_Data.Data_Transfer[16],0,Q5X.Write.BDC[2].Delay_Time_2,16,8)BTD(Port_Data.Data_Transfer[17],0,Q5X.Write.BDC[2].Delay_Time_2,8,8)BTD(Port_Data.Data_Transfer[18],0,Q5X.Write.BDC[2].Delay_Time_2,0,8)BTD(Port_Data.Data_Transfer[19],0,Q5X.Write.BDC[2].Delay_Time_1,24,8)BTD(Port_Data.Data_Transfer[20],0,Q5X.Write.BDC[2].Delay_Time_1,16,8)BTD(Port_Data.Data_Transfer[21],0,Q5X.Write.BDC[2].Delay_Time_1,8,8)BTD(Port_Data.Data_Transfer[22],0,Q5X.Write.BDC[2].Delay_Time_1,0,8)BTD(Port_Data.Data_Transfer[23],0,Q5X.Write.BDC[2].Delay_Mode,0,8)OTU(Port_Data.Port_Read.[Port])OTL(Local_Control.6);
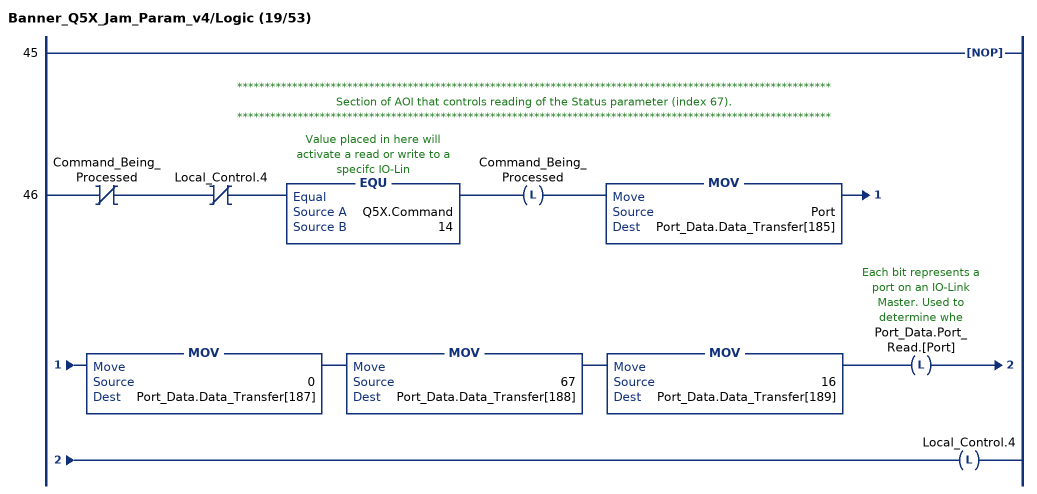
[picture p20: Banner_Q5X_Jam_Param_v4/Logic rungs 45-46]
   45: NOP();
   // ************************************************************************************************************
   // Section of AOI that controls reading of the Status parameter (index 67).
   // ************************************************************************************************************
   46: XIO(Command_Being_Processed)XIO(Local_Control.4)EQU(Q5X.Command,14)OTL(Command_Being_Processed)MOV(Port,Port_Data.Data_Transfer[185])MOV(0,Port_Data.Data_Transfer[187])MOV(67,Port_Data.Data_Transfer[188])MOV(16,Port_Data.Data_Transfer[189])OTL(Port_Data.Port_Read.[Port])OTL(Local_Control.4);
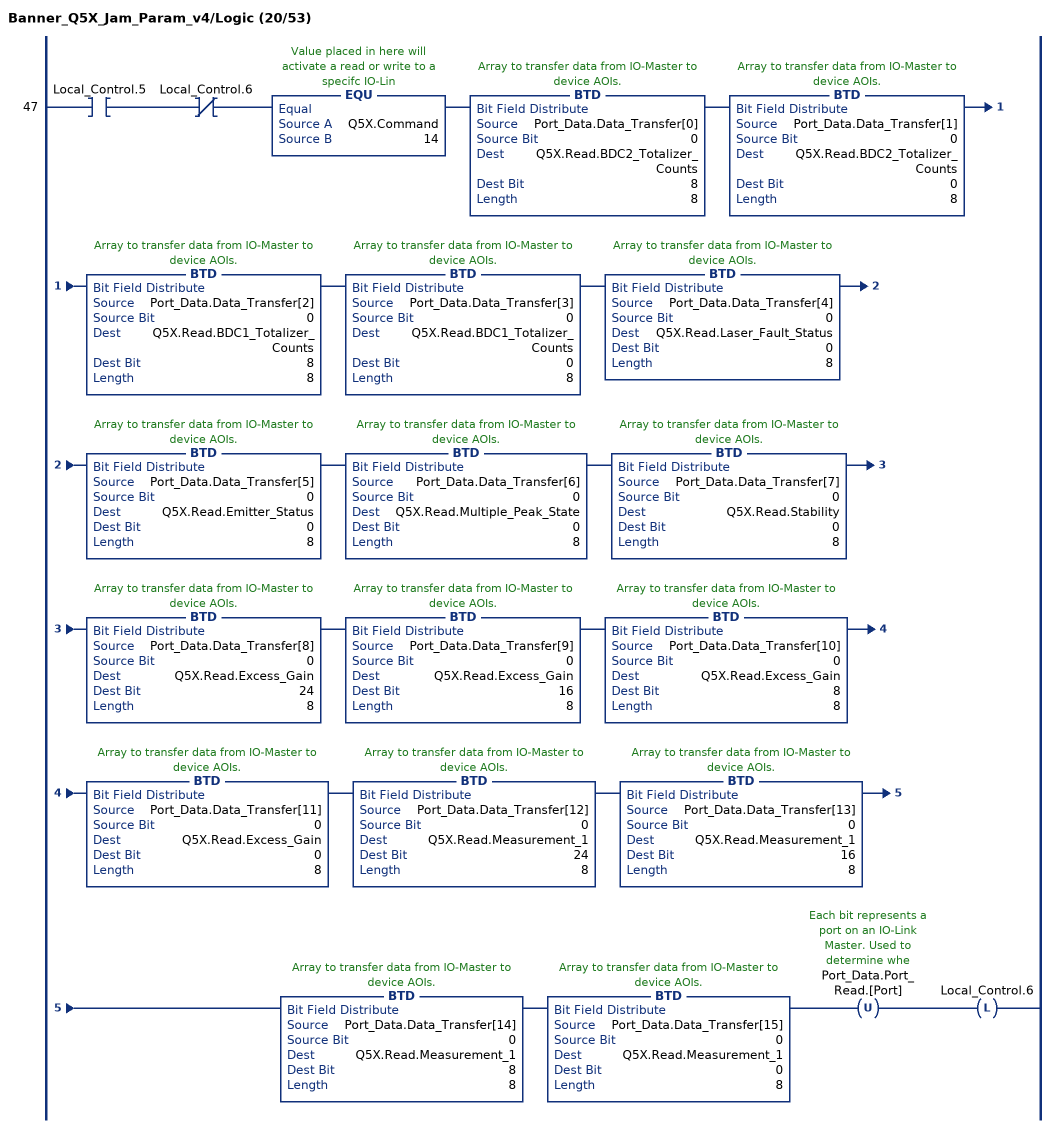
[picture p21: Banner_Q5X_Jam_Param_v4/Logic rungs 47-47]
   47: XIC(Local_Control.5)XIO(Local_Control.6)EQU(Q5X.Command,14)BTD(Port_Data.Data_Transfer[0],0,Q5X.Read.BDC2_Totalizer_Counts,8,8)BTD(Port_Data.Data_Transfer[1],0,Q5X.Read.BDC2_Totalizer_Counts,0,8)BTD(Port_Data.Data_Transfer[2],0,Q5X.Read.BDC1_Totalizer_Counts,8,8)BTD(Port_Data.Data_Transfer[3],0,Q5X.Read.BDC1_Totalizer_Counts,0,8)BTD(Port_Data.Data_Transfer[4],0,Q5X.Read.Laser_Fault_Status,0,8)BTD(Port_Data.Data_Transfer[5],0,Q5X.Read.Emitter_Status,0,8)BTD(Port_Data.Data_Transfer[6],0,Q5X.Read.Multiple_Peak_State,0,8)BTD(Port_Data.Data_Transfer[7],0,Q5X.Read.Stability,0,8)BTD(Port_Data.Data_Transfer[8],0,Q5X.Read.Excess_Gain,24,8)BTD(Port_Data.Data_Transfer[9],0,Q5X.Read.Excess_Gain,16,8)BTD(Port_Data.Data_Transfer[10],0,Q5X.Read.Excess_Gain,8,8)BTD(Port_Data.Data_Transfer[11],0,Q5X.Read.Excess_Gain,0,8)BTD(Port_Data.Data_Transfer[12],0,Q5X.Read.Measurement_1,24,8)BTD(Port_Data.Data_Transfer[13],0,Q5X.Read.Measurement_1,16,8)BTD(Port_Data.Data_Transfer[14],0,Q5X.Read.Measurement_1,8,8)BTD(Port_Data.Data_Transfer[15],0,Q5X.Read.Measurement_1,0,8)OTU(Port_Data.Port_Read.[Port])OTL(Local_Control.6);
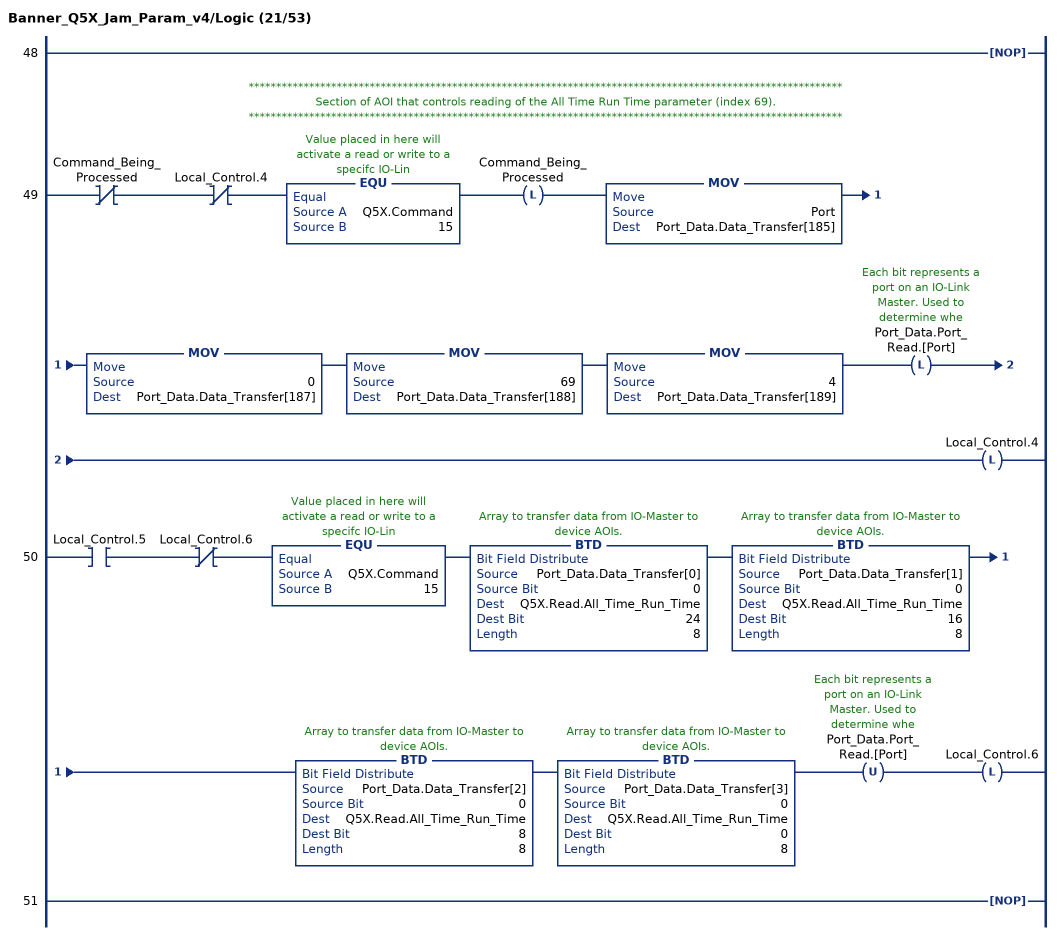
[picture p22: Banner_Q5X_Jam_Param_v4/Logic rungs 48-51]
   48: NOP();
   // ************************************************************************************************************
   // Section of AOI that controls reading of the All Time Run Time parameter (index 69).
   // ************************************************************************************************************
   49: XIO(Command_Being_Processed)XIO(Local_Control.4)EQU(Q5X.Command,15)OTL(Command_Being_Processed)MOV(Port,Port_Data.Data_Transfer[185])MOV(0,Port_Data.Data_Transfer[187])MOV(69,Port_Data.Data_Transfer[188])MOV(4,Port_Data.Data_Transfer[189])OTL(Port_Data.Port_Read.[Port])OTL(Local_Control.4);
   50: XIC(Local_Control.5)XIO(Local_Control.6)EQU(Q5X.Command,15)BTD(Port_Data.Data_Transfer[0],0,Q5X.Read.All_Time_Run_Time,24,8)BTD(Port_Data.Data_Transfer[1],0,Q5X.Read.All_Time_Run_Time,16,8)BTD(Port_Data.Data_Transfer[2],0,Q5X.Read.All_Time_Run_Time,8,8)BTD(Port_Data.Data_Transfer[3],0,Q5X.Read.All_Time_Run_Time,0,8)OTU(Port_Data.Port_Read.[Port])OTL(Local_Control.6);
   51: NOP();
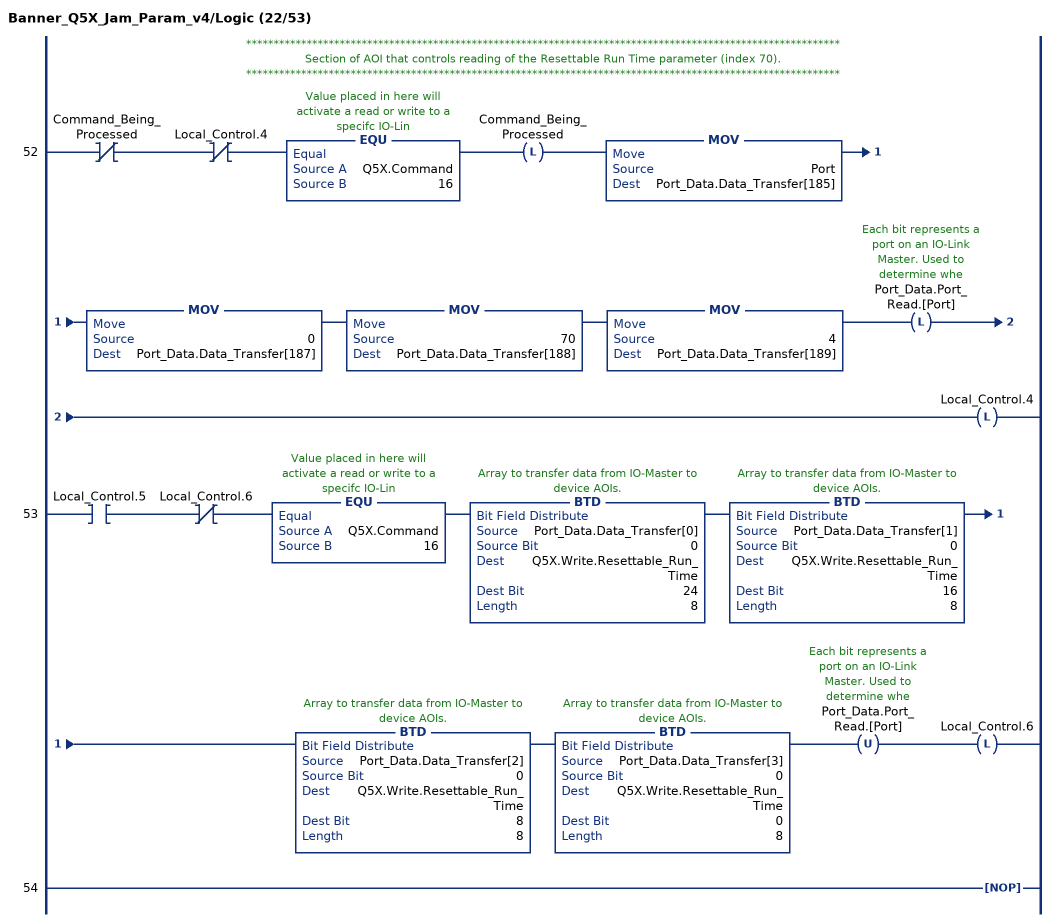
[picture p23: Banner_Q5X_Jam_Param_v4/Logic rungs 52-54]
   // ************************************************************************************************************
   // Section of AOI that controls reading of the Resettable Run Time parameter (index 70).
   // ************************************************************************************************************
   52: XIO(Command_Being_Processed)XIO(Local_Control.4)EQU(Q5X.Command,16)OTL(Command_Being_Processed)MOV(Port,Port_Data.Data_Transfer[185])MOV(0,Port_Data.Data_Transfer[187])MOV(70,Port_Data.Data_Transfer[188])MOV(4,Port_Data.Data_Transfer[189])OTL(Port_Data.Port_Read.[Port])OTL(Local_Control.4);
   53: XIC(Local_Control.5)XIO(Local_Control.6)EQU(Q5X.Command,16)BTD(Port_Data.Data_Transfer[0],0,Q5X.Write.Resettable_Run_Time,24,8)BTD(Port_Data.Data_Transfer[1],0,Q5X.Write.Resettable_Run_Time,16,8)BTD(Port_Data.Data_Transfer[2],0,Q5X.Write.Resettable_Run_Time,8,8)BTD(Port_Data.Data_Transfer[3],0,Q5X.Write.Resettable_Run_Time,0,8)OTU(Port_Data.Port_Read.[Port])OTL(Local_Control.6);
   54: NOP();
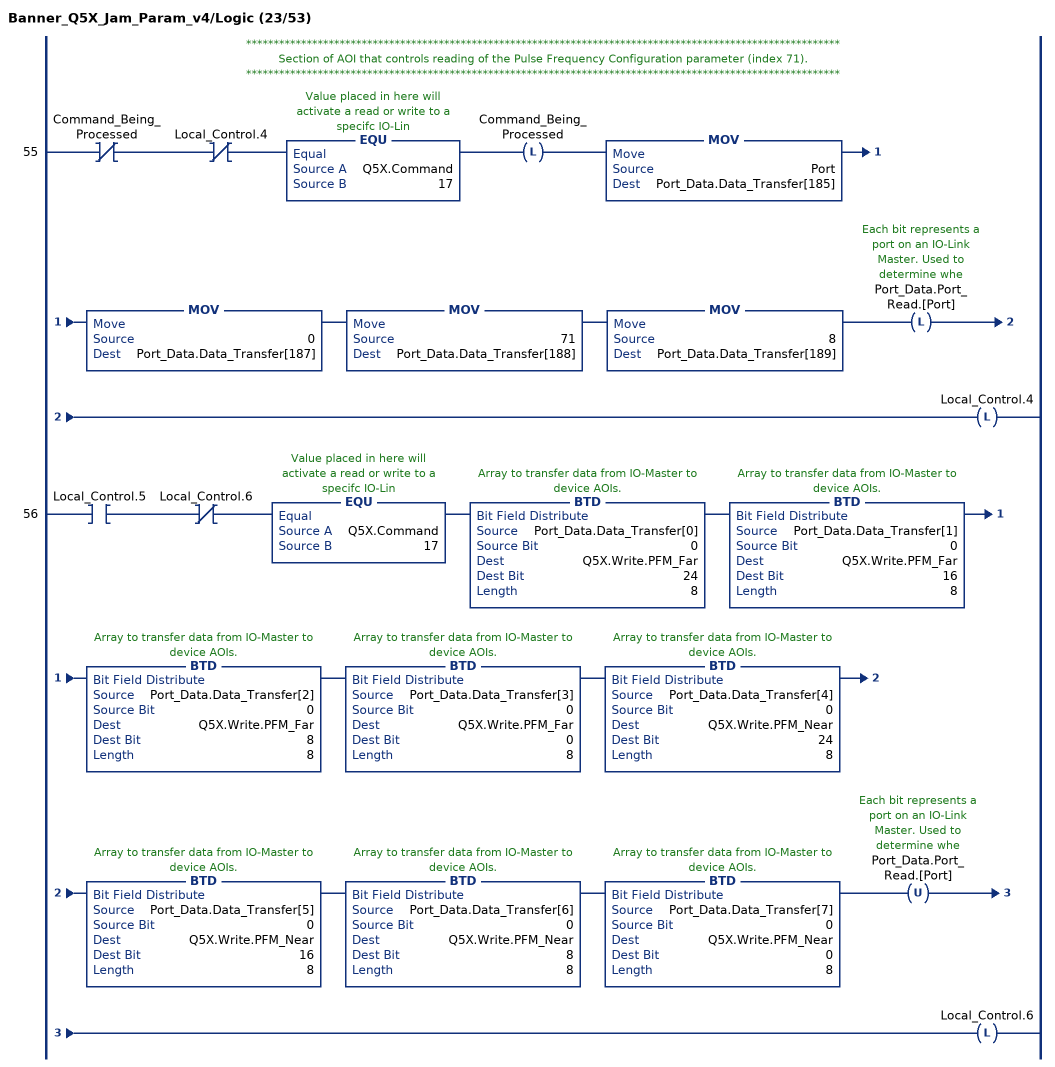
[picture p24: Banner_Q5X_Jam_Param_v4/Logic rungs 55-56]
   // ************************************************************************************************************
   // Section of AOI that controls reading of the Pulse Frequency Configuration parameter (index 71).
   // ************************************************************************************************************
   55: XIO(Command_Being_Processed)XIO(Local_Control.4)EQU(Q5X.Command,17)OTL(Command_Being_Processed)MOV(Port,Port_Data.Data_Transfer[185])MOV(0,Port_Data.Data_Transfer[187])MOV(71,Port_Data.Data_Transfer[188])MOV(8,Port_Data.Data_Transfer[189])OTL(Port_Data.Port_Read.[Port])OTL(Local_Control.4);
   56: XIC(Local_Control.5)XIO(Local_Control.6)EQU(Q5X.Command,17)BTD(Port_Data.Data_Transfer[0],0,Q5X.Write.PFM_Far,24,8)BTD(Port_Data.Data_Transfer[1],0,Q5X.Write.PFM_Far,16,8)BTD(Port_Data.Data_Transfer[2],0,Q5X.Write.PFM_Far,8,8)BTD(Port_Data.Data_Transfer[3],0,Q5X.Write.PFM_Far,0,8)BTD(Port_Data.Data_Transfer[4],0,Q5X.Write.PFM_Near,24,8)BTD(Port_Data.Data_Transfer[5],0,Q5X.Write.PFM_Near,16,8)BTD(Port_Data.Data_Transfer[6],0,Q5X.Write.PFM_Near,8,8)BTD(Port_Data.Data_Transfer[7],0,Q5X.Write.PFM_Near,0,8)OTU(Port_Data.Port_Read.[Port])OTL(Local_Control.6);
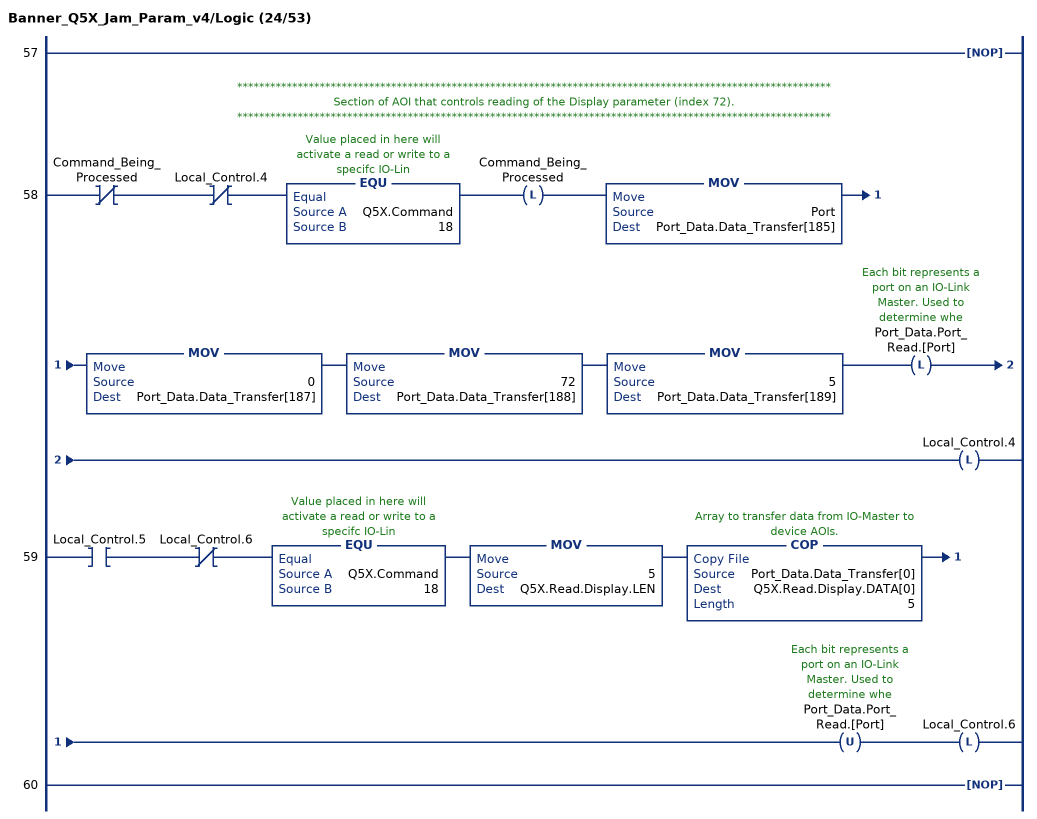
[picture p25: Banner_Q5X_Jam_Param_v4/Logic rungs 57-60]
   57: NOP();
   // ************************************************************************************************************
   // Section of AOI that controls reading of the Display parameter (index 72).
   // ************************************************************************************************************
   58: XIO(Command_Being_Processed)XIO(Local_Control.4)EQU(Q5X.Command,18)OTL(Command_Being_Processed)MOV(Port,Port_Data.Data_Transfer[185])MOV(0,Port_Data.Data_Transfer[187])MOV(72,Port_Data.Data_Transfer[188])MOV(5,Port_Data.Data_Transfer[189])OTL(Port_Data.Port_Read.[Port])OTL(Local_Control.4);
   59: XIC(Local_Control.5)XIO(Local_Control.6)EQU(Q5X.Command,18)MOV(5,Q5X.Read.Display.LEN)COP(Port_Data.Data_Transfer[0],Q5X.Read.Display.DATA[0],5)OTU(Port_Data.Port_Read.[Port])OTL(Local_Control.6);
   60: NOP();
